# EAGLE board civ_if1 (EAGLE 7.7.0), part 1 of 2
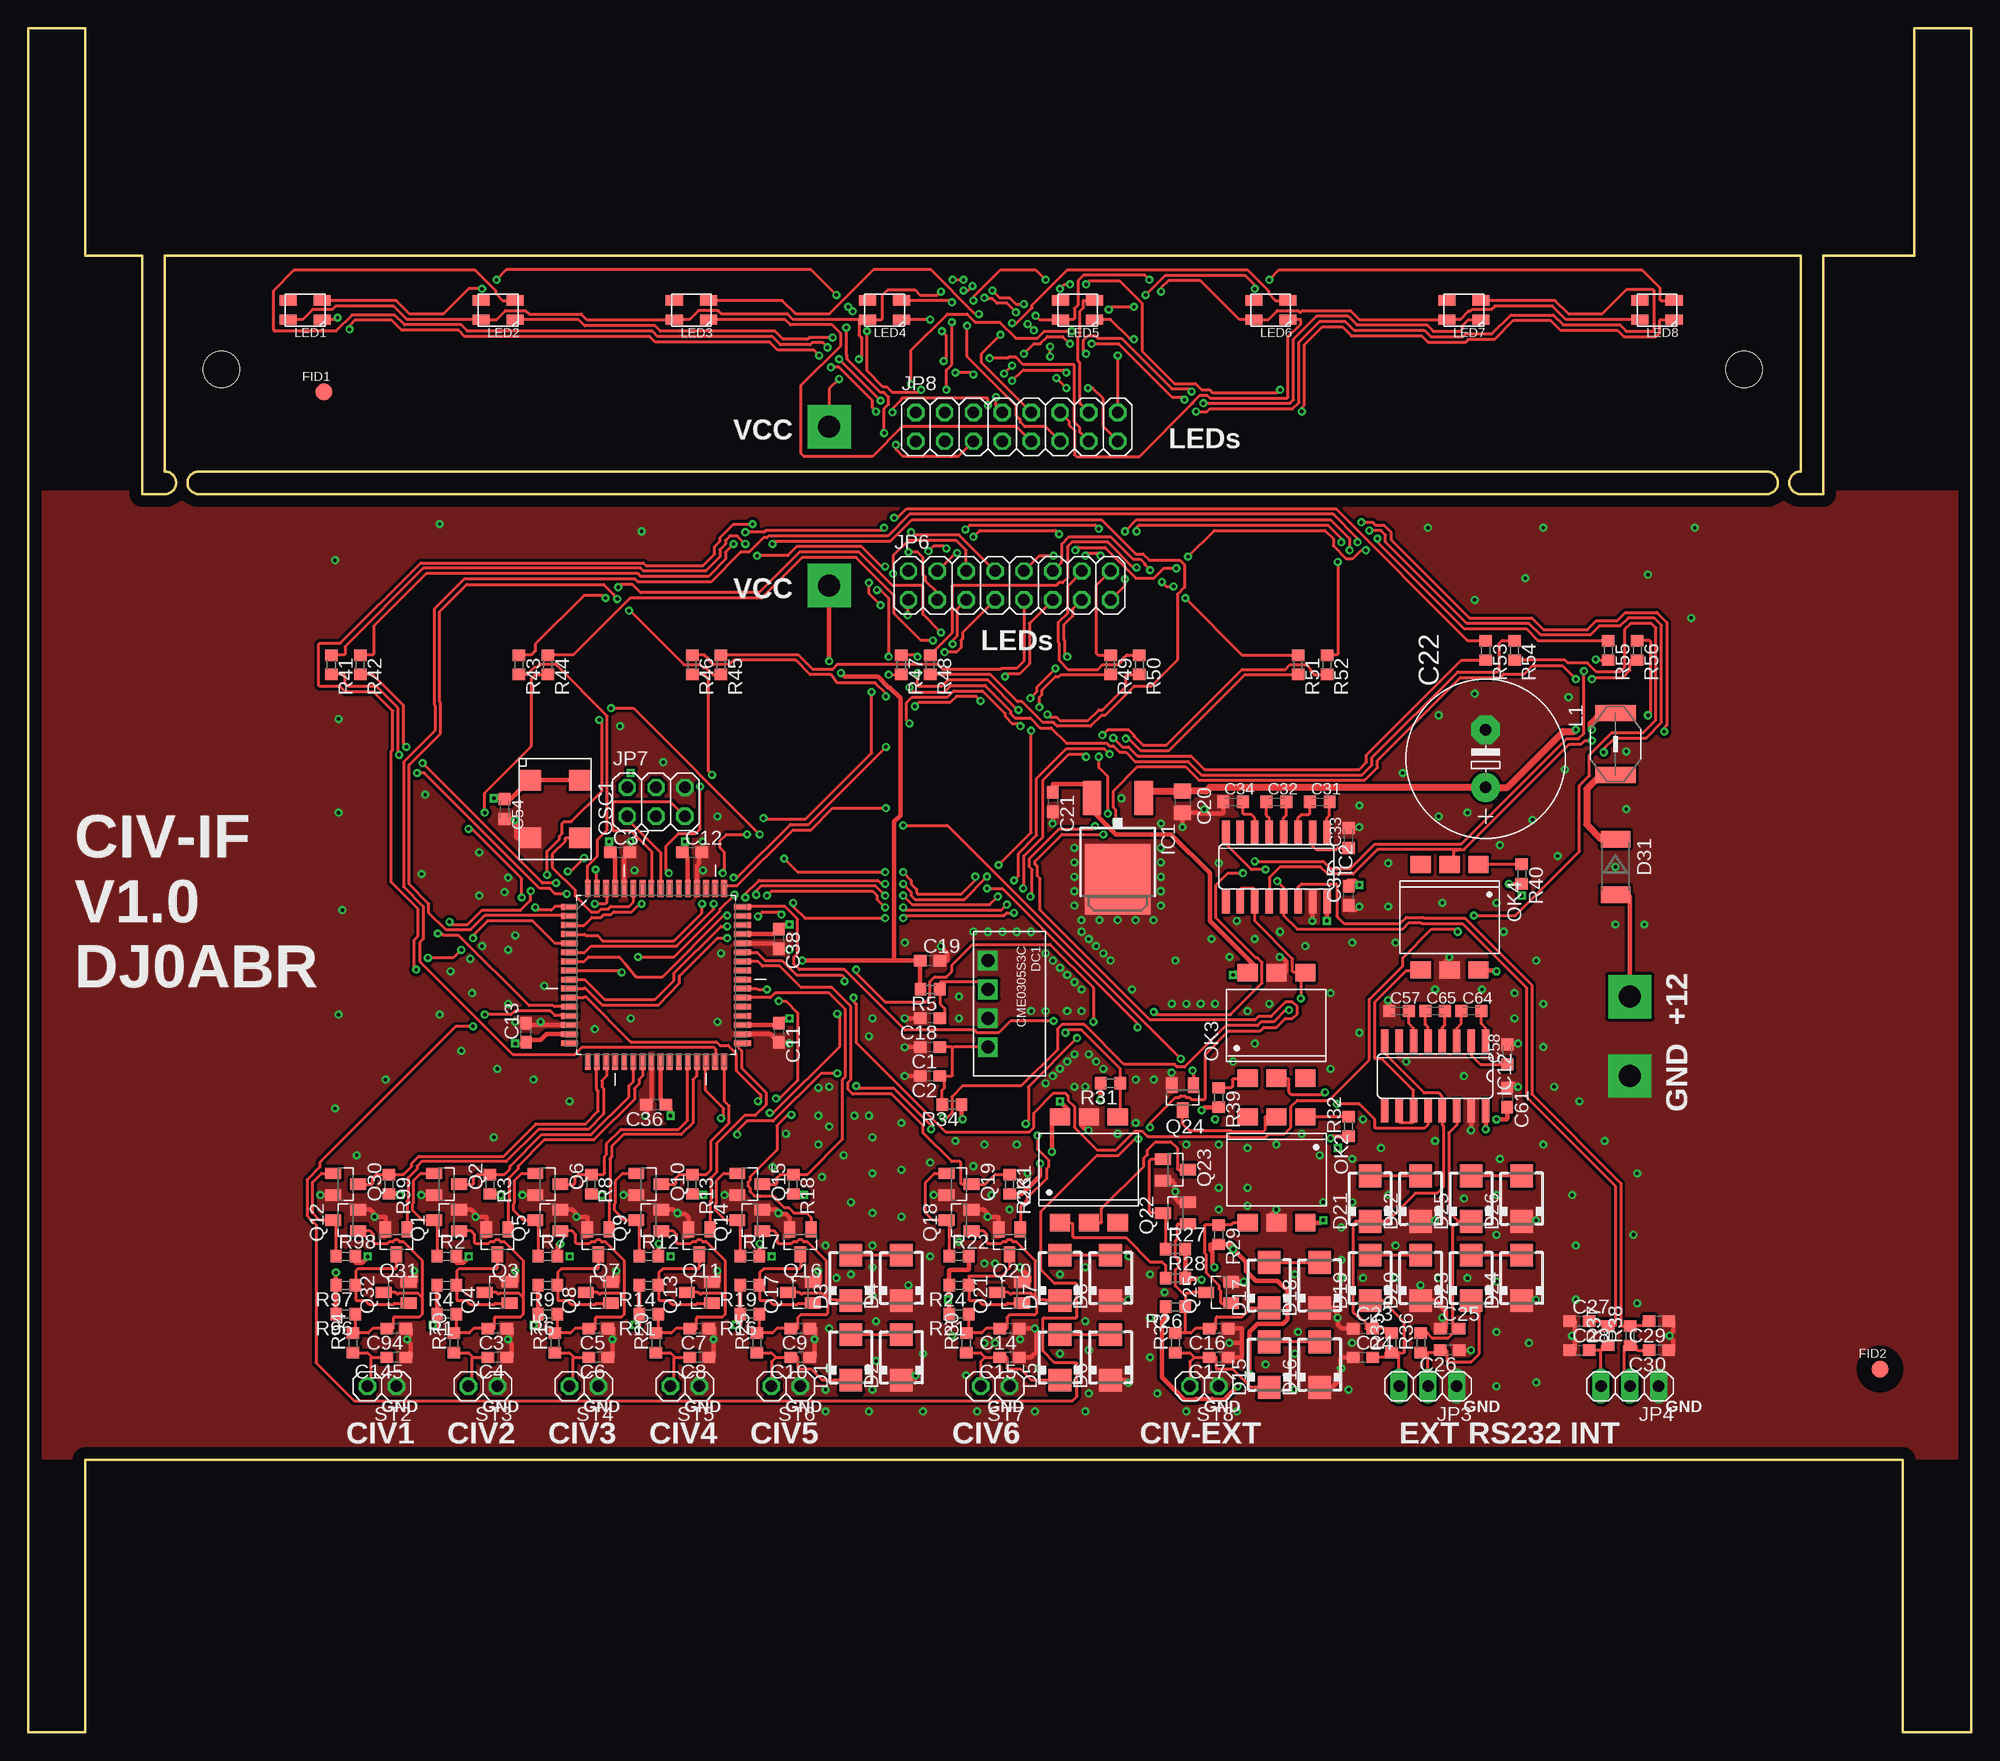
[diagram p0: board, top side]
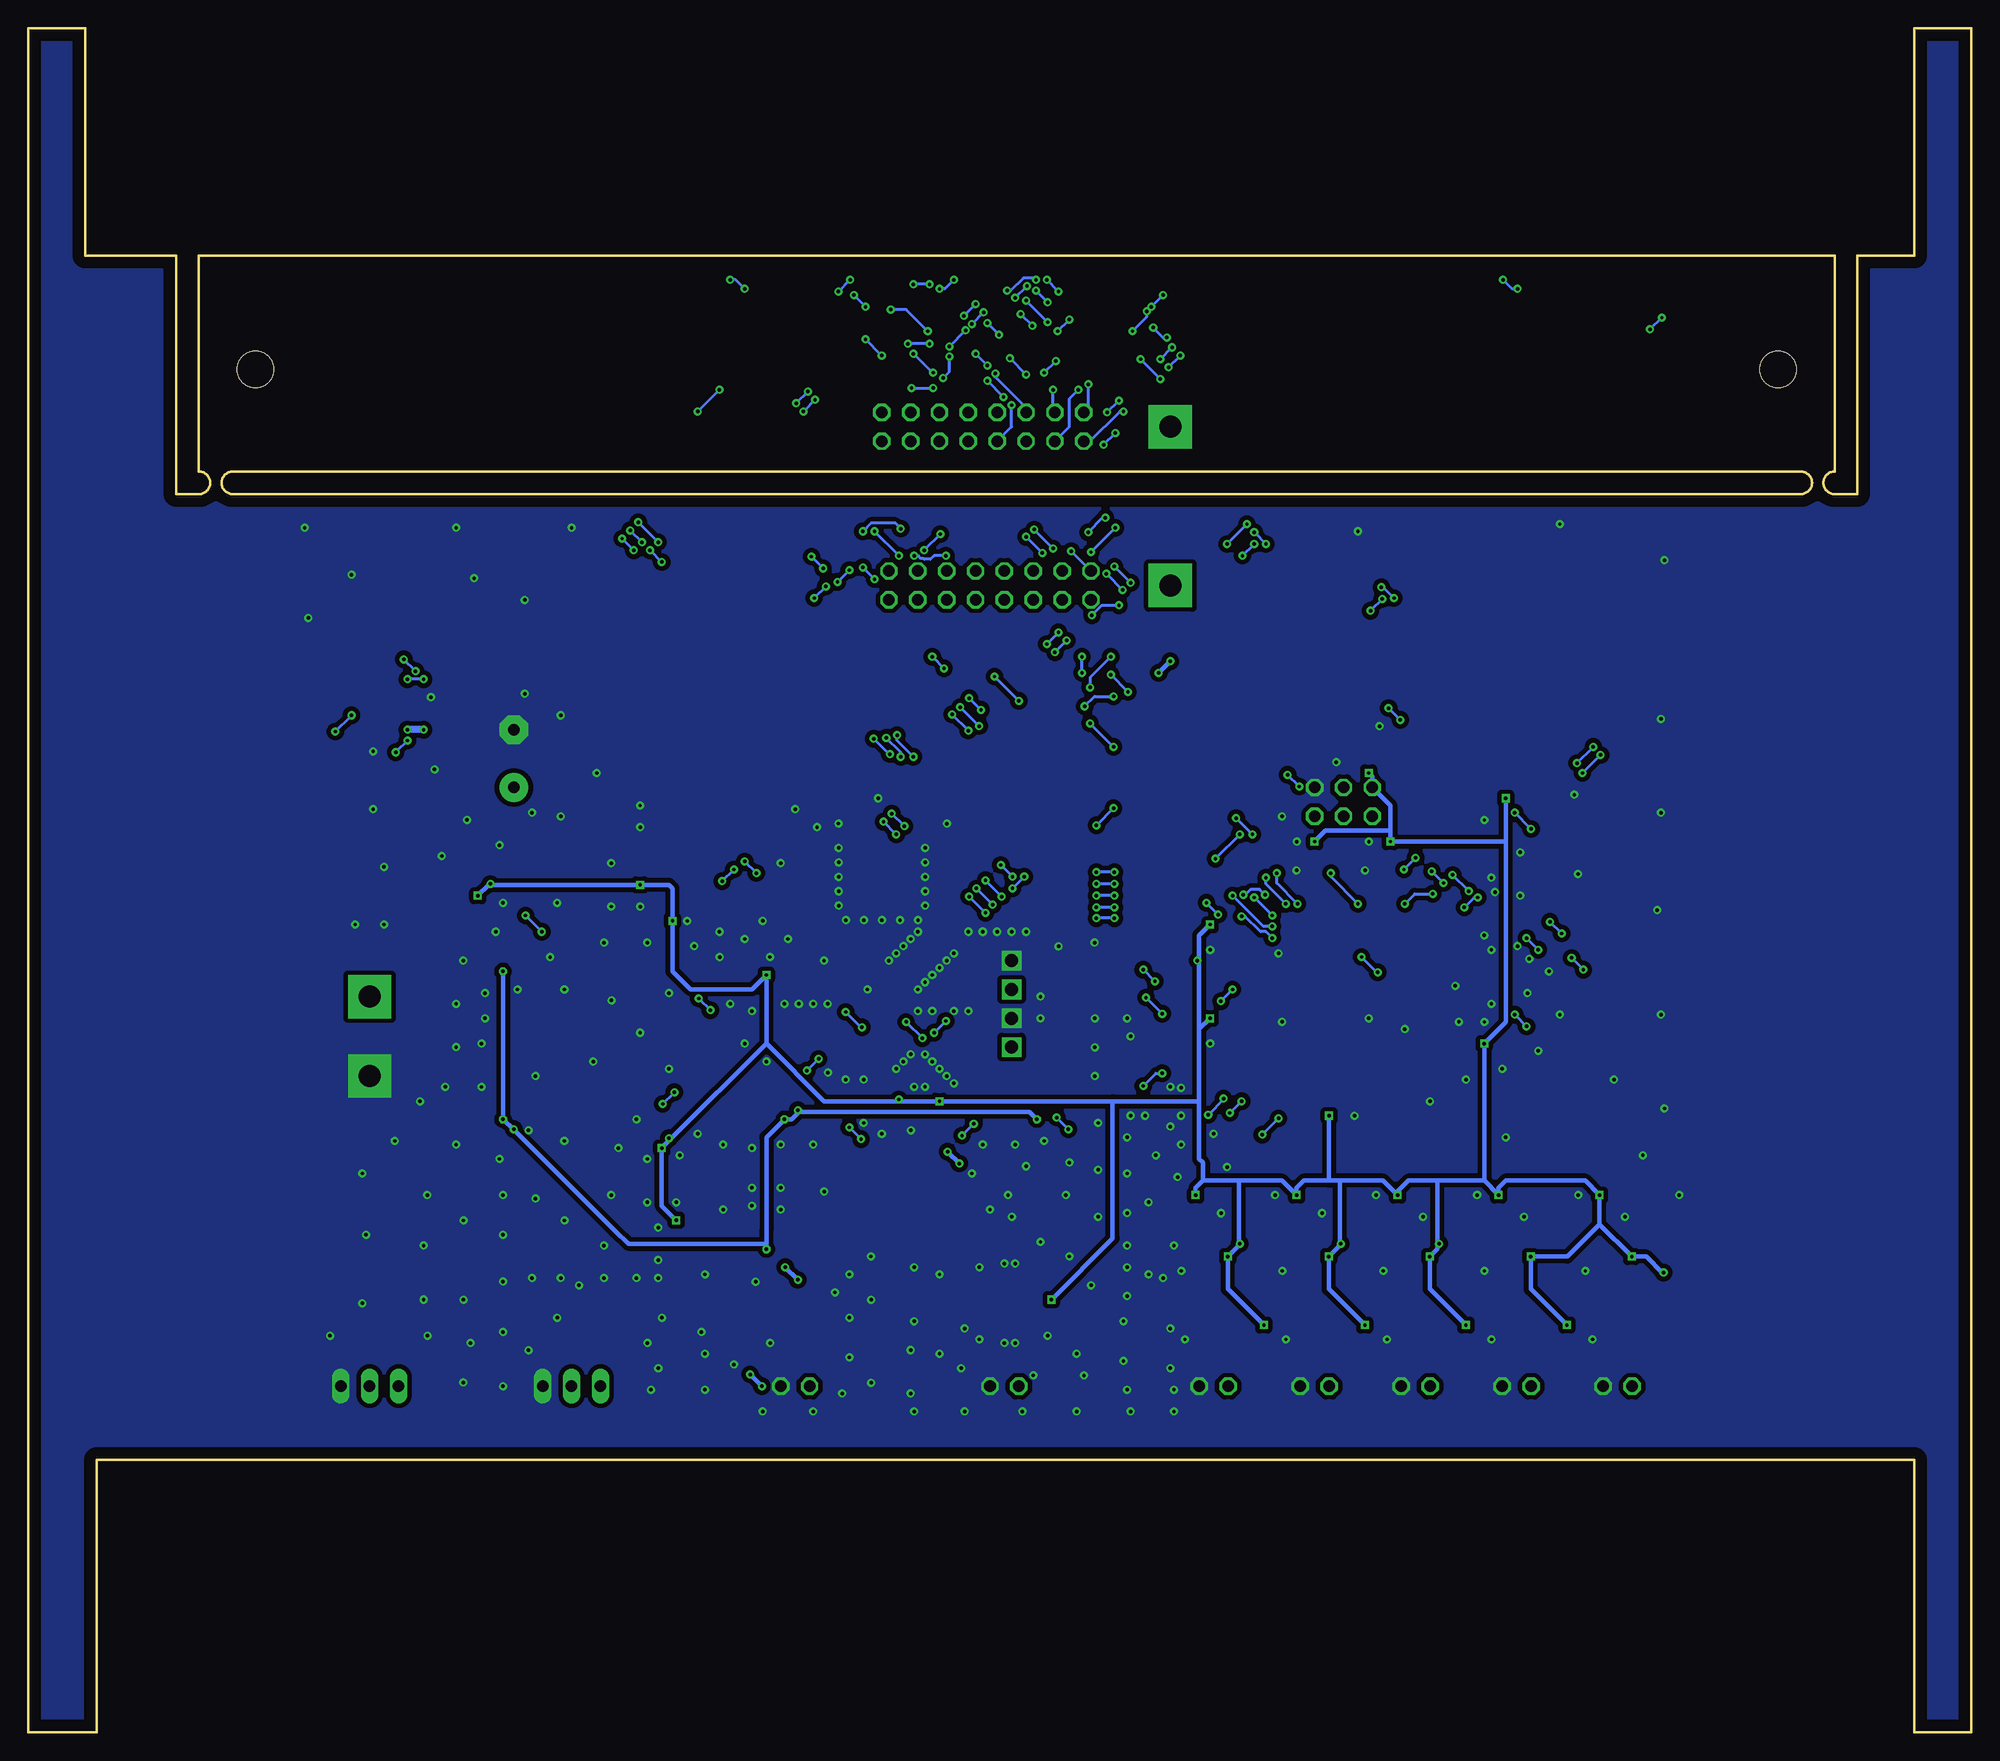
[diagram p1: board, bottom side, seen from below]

Size 171 x 150 mm. Coordinates in mm from the lower left corner, seen from the top.
Outline: 0,0 5,0 5,24 165,24 165,0 171,0 171,150 166,150 166,130 158,130 158,109 156,109 arc-180 156,111 156,130 12,130 12,111 arc-180 12,109 10,109 10,130 5,130 5,150 0,150 0,0
Outline: 153,111 15,111 arc180 15,109 153,109 arc180 153,111
Copper layers (1*16): Top 0.035mm / dielectric 1.5mm / Bottom 0.035mm
Design rules "default *": minimum track width 10mil, minimum drill 0.3mm, track to track 8mil, track to pad 8mil, pad to pad 8mil, via to via 8mil, smd to smd 0mil, copper to edge 40mil, drill to drill 8mil, minimum pad ring 10mil, minimum via ring 8mil, stop-mask expansion 4mil, vias tented up to drill 0.31mm, thermal gap 10mil
Net classes: 1 Supply: width 0.406 mm, drill 0.3 mm; 2 v12: width 0.61 mm, drill 0.3 mm
Holes 3.2 mm at 17,120 151,120

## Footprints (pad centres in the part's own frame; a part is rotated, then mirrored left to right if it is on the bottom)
C0603 = smd 1.1 x 1: 1 -0.85,0; 2 0.85,0
C0805 = smd 1.3 x 1.5: 1 -0.95,0; 2 0.95,0
E5-13 = drill 1.016 pad 2.54: + -2.54,0 | drill 1.016 pad 2.54 octagon: - 2.54,0
C0603K = smd 1.05 x 1.08: 1 -0.875,0; 2 0.875,0
SMA = smd 2 x 2: A 2,0; C -2,0
MELF = smd 1.45 x 2.6: 1 -2.445,0; 2 2.445,0
MURATA_DCDC = drill 1.15 square: 1 -3.81,0; 2 -1.27,0; 3 1.27,0; 4 3.81,0
FIDUCIAL = smd 1.5 x 1.5: P$1 0,0
DPACK = smd 1.6 x 3: 1 -2.28,-4.8; 3 2.28,-4.8 | smd 5.8 x 6.2: 4 0,2.38
SO16 = smd 0.66 x 2.032: 1 -4.445,-3.073; 2 -3.175,-3.073; 3 -1.905,-3.073; 4 -0.635,-3.073; 5 0.635,-3.073; 6 1.905,-3.073; 7 3.175,-3.073; 8 4.445,-3.073; 9 4.445,3.073; 10 3.175,3.073; 11 1.905,3.073; 12 0.635,3.073; 13 -0.635,3.073; 14 -1.905,3.073; 15 -3.175,3.073; 16 -4.445,3.073
THICKPIN = drill 1.93 pad 3.81 square: 1 0,0
1X03 = drill 1.016 long: 1 -2.54,0; 2 0,0; 3 2.54,0
2X08 = drill 1.016 octagon: 1 -8.89,-1.27; 2 -8.89,1.27; 3 -6.35,-1.27; 4 -6.35,1.27; 5 -3.81,-1.27; 6 -3.81,1.27; 7 -1.27,-1.27; 8 -1.27,1.27; 9 1.27,-1.27; 10 1.27,1.27; 11 3.81,-1.27; 12 3.81,1.27; 13 6.35,-1.27; 14 6.35,1.27; 15 8.89,-1.27; 16 8.89,1.27
2X03 = drill 1.016 octagon: 1 -2.54,-1.27; 2 -2.54,1.27; 3 0,-1.27; 4 0,1.27; 5 2.54,-1.27; 6 2.54,1.27
S = smd 1.4 x 3.56: 1 -2.73,0; 2 2.73,0
PLCC4_WE_LED = smd 1.5 x 0.9: 1 1.51,0.88; 2 1.51,-0.82; 3 -1.49,0.88; 4 -1.49,-0.82
DIL6-SMD = smd 1.78 x 1.52: 1 -2.54,-4.645; 2 0,-4.645; 3 2.54,-4.645; 4 2.54,4.645; 5 0,4.645; 6 -2.54,4.645
QOSC_AQO7015 = smd 1.8 x 2: 1 0,-0.318; 2 5.08,-0.318; 3 5.08,4.128; 4 0,4.128
SOT23 = smd 1 x 1.4: 1 -0.95,-1.1; 2 0.95,-1.1; 3 0,1.1
R0603 = smd 1 x 1.1: 1 -0.85,0; 2 0.85,0
PINHEAD1X2 = drill 1.016 octagon: 1 -1.27,0; 2 1.27,0
QFP80P1600X1600X120-64N = smd 1.473 x 0.508: 1 -7.62,5.994; 2 -7.62,5.207; 3 -7.62,4.394; 4 -7.62,3.607; 5 -7.62,2.794; 6 -7.62,2.007; 7 -7.62,1.194; 8 -7.62,0.406; 9 -7.62,-0.406; 10 -7.62,-1.194; 11 -7.62,-2.007; 12 -7.62,-2.794; 13 -7.62,-3.607; 14 -7.62,-4.394; 15 -7.62,-5.207; 16 -7.62,-5.994; 33 7.62,-5.994; 34 7.62,-5.207; 35 7.62,-4.394; 36 7.62,-3.607; 37 7.62,-2.794; 38 7.62,-2.007; 39 7.62,-1.194; 40 7.62,-0.406; 41 7.62,0.406; 42 7.62,1.194; 43 7.62,2.007; 44 7.62,2.794; 45 7.62,3.607; 46 7.62,4.394; 47 7.62,5.207; 48 7.62,5.994 | smd 0.508 x 1.473: 17 -5.994,-7.62; 18 -5.207,-7.62; 19 -4.394,-7.62; 20 -3.607,-7.62; 21 -2.794,-7.62; 22 -2.007,-7.62; 23 -1.194,-7.62; 24 -0.406,-7.62; 25 0.406,-7.62; 26 1.194,-7.62; 27 2.007,-7.62; 28 2.794,-7.62; 29 3.607,-7.62; 30 4.394,-7.62; 31 5.207,-7.62; 32 5.994,-7.62; 49 5.994,7.62; 50 5.207,7.62; 51 4.394,7.62; 52 3.607,7.62; 53 2.794,7.62; 54 2.007,7.62; 55 1.194,7.62; 56 0.406,7.62; 57 -0.406,7.62; 58 -1.194,7.62; 59 -2.007,7.62; 60 -2.794,7.62; 61 -3.607,7.62; 62 -4.394,7.62; 63 -5.207,7.62; 64 -5.994,7.62

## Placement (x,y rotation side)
C1  100n  [C0603]  79.38,60.33 180 top
C2  1u  [C0603]  79.38,57.78 180 top
C3  1n  [C0603]  41.27,35.56 180 top
C4  1n  [C0603]  41.27,33.02 180 top
C5  1n  [C0603]  50.16,35.56 180 top
C6  1n  [C0603]  50.16,33.02 180 top
C7  1n  [C0603]  59.05,35.56 180 top
C8  1n  [C0603]  59.05,33.02 180 top
C9  1n  [C0603]  67.94,35.56 180 top
C10  1n  [C0603]  67.94,33.02 180 top
C11  100n  [C0603]  66.04,61.59 270 top
C12  100n  [C0603]  58.42,77.47 0 top
C13  1u  [C0603]  43.81,61.59 90 top
C14  1n  [C0603]  86.36,35.56 180 top
C15  1n  [C0603]  86.36,33.02 180 top
C16  100p  [C0603]  104.78,35.56 180 top
C17  100p  [C0603]  104.78,33.02 180 top
C18  1u  [C0603]  79.38,62.87 180 top
C19  1u  [C0603]  79.38,67.94 0 top
C20  10u  [C0805]  101.6,81.92 270 top
C21  10u  [C0603]  90.17,81.92 270 top
C22  1000u/16  [E5-13]  128.27,85.72 90 top
C23  100p  [C0603]  117.47,35.56 0 top
C24  100p  [C0603]  117.47,33.02 0 top
C25  100p  [C0603]  125.09,35.56 0 top
C26  100p  [C0603]  125.09,33.66 180 top
C27  1n  [C0603]  136.53,36.2 0 top
C28  1n  [C0603]  136.53,33.66 0 top
C29  1n  [C0603]  143.51,36.2 180 top
C30  1n  [C0603]  143.51,33.66 180 top
C31  1u  [C0603K]  113.67,81.92 0 top
C32  1u  [C0603K]  109.86,81.92 0 top
C33  1u  [C0603K]  116.2,78.74 90 top
C34  1u  [C0603K]  106.05,81.92 0 top
C35  1u  [C0603]  116.2,73.66 90 top
C36  100n  [C0603]  55.24,55.24 180 top
C37  100n  [C0603]  52.07,77.47 0 top
C38  1u  [C0603]  66.04,69.85 270 top
C54  1u  [C0603K]  41.91,81.28 270 top
C57  1u  [C0603K]  120.65,63.5 0 top
C58  1u  [C0603K]  130.18,59.69 90 top
C61  1u  [C0603]  130.18,55.88 270 top
C64  1u  [C0603K]  127,63.5 0 top
C65  1u  [C0603K]  123.83,63.5 0 top
C94  1n  [C0603]  32.38,35.56 180 top
C145  1n  [C0603]  32.38,33.02 180 top
D1  SMBJ15A  [SMA]  72.39,33.02 90 top
D2  SMBJ15A  [SMA]  76.83,33.02 90 top
D3  SMBJ15A  [SMA]  72.39,40.01 90 top
D4  SMBJ15A  [SMA]  76.83,40.01 90 top
D5  SMBJ15A  [SMA]  90.81,33.02 90 top
D6  SMBJ15A  [SMA]  95.25,33.02 90 top
D7  SMBJ15A  [SMA]  90.81,40.01 90 top
D8  SMBJ15A  [SMA]  95.25,40.01 90 top
D15  SMBJ15A  [SMA]  109.22,32.38 90 top
D16  SMBJ15A  [SMA]  113.67,32.38 90 top
D17  SMBJ15A  [SMA]  109.22,39.37 90 top
D18  SMBJ15A  [SMA]  113.67,39.37 90 top
D19  SMBJ15A  [SMA]  118.11,40.01 90 top
D20  SMBJ15A  [SMA]  122.56,40.01 90 top
D21  SMBJ15A  [SMA]  118.11,46.99 90 top
D22  SMBJ15A  [SMA]  122.56,46.99 90 top
D23  SMBJ15A  [SMA]  127,40.01 90 top
D24  SMBJ15A  [SMA]  131.44,40.01 90 top
D25  SMBJ15A  [SMA]  127,46.99 90 top
D26  SMBJ15A  [SMA]  131.44,46.99 90 top
D31  1N4001  [MELF]  139.7,76.2 270 top
DC1  CME0305S3C  [MURATA_DCDC]  84.45,64.14 270 top
FID1  FIDUCIAL  [FIDUCIAL]  26,118 0 top
FID2  FIDUCIAL  [FIDUCIAL]  163,32 0 top
IC1  LF33CDT-DPAK  [DPACK]  95.89,77.47 180 top
IC2  MAX3232  [SO16]  109.86,76.2 180 top
IC12  MAX3232  [SO16]  123.83,57.78 180 top
JP1  [THICKPIN]  140.97,64.77 90 top
JP2  [THICKPIN]  140.97,57.78 90 top
JP3  [1X03]  123.19,30.48 180 top
JP4  [1X03]  140.97,30.48 180 top
JP5  [THICKPIN]  70.48,100.97 0 top
JP6  [2X08]  86.36,100.97 0 top
JP7  Program  [2X03]  55.24,81.92 0 top
JP8  [2X08]  87,114.94 0 top
JP9  [THICKPIN]  70.48,114.94 0 top
L1  WE74451147/47uH  [S]  139.7,87 270 top
LED1  RGBLED  [PLCC4_WE_LED]  24.36,125.24 180 top
LED2  RGBLED  [PLCC4_WE_LED]  41.37,125.24 180 top
LED3  RGBLED  [PLCC4_WE_LED]  58.37,125.24 180 top
LED4  RGBLED  [PLCC4_WE_LED]  75.36,125.24 180 top
LED5  RGBLED  [PLCC4_WE_LED]  92.36,125.24 180 top
LED6  RGBLED  [PLCC4_WE_LED]  109.36,125.24 180 top
LED7  RGBLED  [PLCC4_WE_LED]  126.36,125.24 180 top
LED8  RGBLED  [PLCC4_WE_LED]  143.37,125.24 180 top
OK1  H11L1SM  [DIL6-SMD]  93.34,49.53 0 top
OK2  H11L1SM  [DIL6-SMD]  109.86,49.53 180 top
OK3  H11L1SM  [DIL6-SMD]  109.86,62.23 0 top
OK4  H11L1SM  [DIL6-SMD]  125.09,71.75 180 top
OSC1  OSZ8MHz  [QOSC_AQO7015]  44.45,83.82 270 top
Q1  N-CH_MOSFET  [SOT23]  36.83,45.09 90 top
Q2  N-CH_MOSFET  [SOT23]  36.83,48.26 270 top
Q3  N-CH_MOSFET  [SOT23]  41.27,43.18 180 top
Q4  N-CH_MOSFET  [SOT23]  41.27,38.73 90 top
Q5  N-CH_MOSFET  [SOT23]  45.72,45.09 90 top
Q6  N-CH_MOSFET  [SOT23]  45.72,48.26 270 top
Q7  N-CH_MOSFET  [SOT23]  50.16,43.18 180 top
Q8  N-CH_MOSFET  [SOT23]  50.16,38.73 90 top
Q9  N-CH_MOSFET  [SOT23]  54.61,45.09 90 top
Q10  N-CH_MOSFET  [SOT23]  54.61,48.26 270 top
Q11  N-CH_MOSFET  [SOT23]  59.05,43.18 180 top
Q12  N-CH_MOSFET  [SOT23]  27.94,45.09 90 top
Q13  N-CH_MOSFET  [SOT23]  59.05,38.73 90 top
Q14  N-CH_MOSFET  [SOT23]  63.5,45.09 90 top
Q15  N-CH_MOSFET  [SOT23]  63.5,48.26 270 top
Q16  N-CH_MOSFET  [SOT23]  67.94,43.18 180 top
Q17  N-CH_MOSFET  [SOT23]  67.94,38.73 90 top
Q18  N-CH_MOSFET  [SOT23]  81.92,45.09 90 top
Q19  N-CH_MOSFET  [SOT23]  81.92,48.26 270 top
Q20  N-CH_MOSFET  [SOT23]  86.36,43.18 180 top
Q21  N-CH_MOSFET  [SOT23]  86.36,38.73 90 top
Q22  N-CH_MOSFET  [SOT23]  100.97,45.72 90 top
Q23  N-CH_MOSFET  [SOT23]  100.97,49.53 270 top
Q24  N-CH_MOSFET  [SOT23]  101.6,55.88 180 top
Q25  N-CH_MOSFET  [SOT23]  104.78,38.73 90 top
Q30  N-CH_MOSFET  [SOT23]  27.94,48.26 270 top
Q31  N-CH_MOSFET  [SOT23]  32.38,43.18 180 top
Q32  N-CH_MOSFET  [SOT23]  32.38,38.73 90 top
R1  10k  [R0603]  36.83,36.83 180 top
R2  10k  [R0603]  36.83,41.91 0 top
R3  10k  [R0603]  40.64,48.26 270 top
R4  10k  [R0603]  36.83,39.37 180 top
R5  1kOhm-Ferr  [R0603]  79.38,65.41 180 top
R6  10k  [R0603]  45.72,36.83 180 top
R7  10k  [R0603]  45.72,41.91 0 top
R8  10k  [R0603]  49.53,48.26 270 top
R9  10k  [R0603]  45.72,39.37 180 top
R10  1kOhm-Ferr  [R0603]  37.47,34.29 90 top
R11  10k  [R0603]  54.61,36.83 180 top
R12  10k  [R0603]  54.61,41.91 0 top
R13  10k  [R0603]  58.42,48.26 270 top
R14  10k  [R0603]  54.61,39.37 180 top
R15  1kOhm-Ferr  [R0603]  46.35,34.29 90 top
R16  10k  [R0603]  63.5,36.83 180 top
R17  10k  [R0603]  63.5,41.91 0 top
R18  10k  [R0603]  67.31,48.26 270 top
R19  10k  [R0603]  63.5,39.37 180 top
R20  1kOhm-Ferr  [R0603]  55.24,34.29 90 top
R21  10k  [R0603]  81.92,36.83 180 top
R22  10k  [R0603]  81.92,41.91 0 top
R23  10k  [R0603]  86.36,48.26 270 top
R24  10k  [R0603]  81.92,39.37 180 top
R25  1kOhm-Ferr  [R0603]  64.14,34.29 90 top
R26  10k  [R0603]  100.97,37.47 180 top
R27  10k  [R0603]  100.97,42.55 0 top
R28  680  [R0603]  100.97,40.01 0 top
R29  1k  [R0603]  104.78,43.81 270 top
R30  1kOhm-Ferr  [R0603]  82.55,34.29 90 top
R31  1k  [R0603]  95.25,57.15 180 top
R32  330  [R0603]  116.2,53.34 90 top
R33  1kOhm-Ferr  [R0603]  100.97,34.29 90 top
R34  1kOhm-Ferr  [R0603]  81.28,55.24 180 top
R35  1kOhm-Ferr  [R0603]  120.02,34.29 90 top
R36  1kOhm-Ferr  [R0603]  122.56,34.29 90 top
R37  1kOhm-Ferr  [R0603]  139.06,34.92 90 top
R38  1kOhm-Ferr  [R0603]  140.97,34.92 90 top
R39  680  [R0603]  104.78,55.88 270 top
R40  330  [R0603]  131.44,75.56 270 top
R41  2k2  [R0603]  26.67,93.98 270 top
R42  680  [R0603]  29.21,93.98 270 top
R43  2k2  [R0603]  43.18,93.98 270 top
R44  680  [R0603]  45.72,93.98 270 top
R45  2k2  [R0603]  60.96,93.98 270 top
R46  680  [R0603]  58.42,93.98 270 top
R47  2k2  [R0603]  76.83,93.98 270 top
R48  680  [R0603]  79.38,93.98 270 top
R49  2k2  [R0603]  95.25,93.98 270 top
R50  680  [R0603]  97.79,93.98 270 top
R51  2k2  [R0603]  111.76,93.98 270 top
R52  680  [R0603]  114.3,93.98 270 top
R53  2k2  [R0603]  128.27,95.25 270 top
R54  680  [R0603]  130.81,95.25 270 top
R55  2k2  [R0603]  139.06,95.25 270 top
R56  680  [R0603]  141.6,95.25 270 top
R94  1kOhm-Ferr  [R0603]  28.57,34.29 90 top
R96  10k  [R0603]  27.94,36.83 180 top
R97  10k  [R0603]  27.94,39.37 180 top
R98  10k  [R0603]  27.94,41.91 0 top
R99  10k  [R0603]  31.75,48.26 270 top
ST2  [PINHEAD1X2]  31.11,30.48 180 top
ST3  [PINHEAD1X2]  40.01,30.48 180 top
ST4  [PINHEAD1X2]  48.9,30.48 180 top
ST5  [PINHEAD1X2]  57.78,30.48 180 top
ST6  [PINHEAD1X2]  66.67,30.48 180 top
ST7  [PINHEAD1X2]  85.09,30.48 180 top
ST8  [PINHEAD1X2]  103.5,30.48 180 top
U1  ATXMEGA256A3-AU  [QFP80P1600X1600X120-64N]  55.24,66.67 0 top

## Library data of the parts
C1-C38 C54 C57 C58 C61 C64 C65 C94 C145 R1-R56 R94 R96-R99 = rcl
D1-D8 D15-D26 D31 DC1 FID1 FID2 JP1 JP2 JP5 JP9 LED1-LED8 OSC1 Q1-Q25 Q30-Q32 ST2-ST8 = km
IC1 = v-reg
IC2 IC12 = maxim; MPN: MAX3232CSE; OC_FARNELL: 9725490; OC_NEWARK: 90C2890
JP3 JP4 JP6-JP8 = pinhead
L1 = WE-PD3; MPN: 74451147; OC_FARNELL: 1636065; OC_NEWARK: 08P2637; PACKAGE: Type S; SUPPLIER: Würth Elektronik eiSos GmbH
OK1-OK4 = optocoupler; OC_FARNELL: unknown; OC_NEWARK: unknown
U1 = ATXMEGA256A3-AU; DESCRIPTION: MCU; MPN: ATXMEGA256A3-AU; OC_FARNELL: 1748554; OC_NEWARK: -; PACKAGE: QFP-64; SUPPLIER: Atmel

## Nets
GND [Supply]: C1.2 C2.2 C3.1 C4.1 C5.1 C6.1 C7.1 C8.1 C9.1 C10.1 C11.2 C12.2 C13.2 C14.1 C15.1 C16.1 C17.1 C18.2 C19.2 C20.2 C21.2 C22.- C23.1 C24.1 C25.1 C26.1 C27.1 C28.1 C29.1 C30.1 C33.2 C34.1 C35.1 C36.2 C37.2 C38.2 C54.2 C57.1 C58.2 C61.1 C94.1 C145.1 D2.C D4.C D6.C D8.C D16.C D18.C D20.C D22.C D24.C D26.C DC1.1 DC1.3 IC1.4 IC2.15 IC12.15 JP2.1 JP3.1 JP4.1 JP7.6 OK1.5 OK2.5 OK3.5 OK4.5 OSC1.2 Q1.2 Q2.2 Q3.2 Q4.2 Q5.2 Q6.2 Q7.2 Q8.2 Q9.2 Q10.2 Q11.2 Q12.2 Q13.2 Q14.2 Q15.2 Q16.2 Q17.2 Q18.2 Q19.2 Q20.2 Q21.2 Q22.2 Q23.2 Q24.2 Q25.2 Q30.2 Q31.2 Q32.2 ST2.1 ST3.1 ST4.1 ST5.1 ST6.1 ST7.1 ST8.1 U1.14 U1.24 U1.34 U1.44 U1.52 U1.60
N$1: OK1.2 Q23.3
N$2: Q1.3 Q2.1 R2.1
N$3: OSC1.3 U1.59
N$4: C1.1 C2.1 DC1.4 R34.2
N$5: Q3.3 Q4.1 R4.1
N$6: C18.1 DC1.2 R5.1
N$7: C4.2 R10.1 ST3.2
N$8: OK2.1 R32.2
N$9: Q5.3 Q6.1 R7.1
N$10: C94.2 Q12.1 Q32.3 R94.2 R96.1
N$11: C3.2 Q1.1 Q4.3 R1.1 R10.2
N$12: Q7.3 Q8.1 R9.1
N$13: C6.2 R15.1 ST4.2
N$14: C5.2 Q5.1 Q8.3 R6.1 R15.2
N$15: C8.2 R20.1 ST5.2
N$16: Q9.3 Q10.1 R12.1
N$17: Q22.3 Q23.1 R27.1
N$18: OK2.4 Q25.1 R29.1
N$19: Q11.3 Q13.1 R14.1
N$20 [v12]: C20.1 C22.+ IC1.1 L1.1
N$21: C7.2 Q9.1 Q13.3 R11.1 R20.2
N$22: C10.2 D1.C R25.1 ST6.2
N$23: Q14.3 Q15.1 R17.1
N$24: C9.2 D3.C Q14.1 Q17.3 R16.1 R25.2
N$25: C15.2 D5.C R30.1 ST7.2
N$26: Q16.3 Q17.1 R19.1
N$27: JP6.1 R41.1
N$28: C14.2 D7.C Q18.1 Q21.3 R21.1 R30.2
N$29: C17.2 D15.C R33.1 ST8.2
N$30: Q18.3 Q19.1 R22.1
N$31: C16.2 D17.C Q22.1 Q25.3 R26.1 R33.2
N$32: JP6.3 R42.1
N$33: Q20.3 Q21.1 R24.1
N$34 [Supply]: D31.2 JP1.1
N$35: D15.A D16.A
N$36: D17.A D18.A
N$37: C24.2 D19.C JP3.3 R35.1
N$38: C23.2 D21.C IC12.8 IC12.13 R35.2
N$39: D19.A D20.A
N$40: D21.A D22.A
N$41: C26.2 D23.C JP3.2 R36.1
N$42: C28.2 JP4.3 R37.1
N$43: D23.A D24.A
N$44: D25.A D26.A
N$45: C64.1 IC12.3
N$46: C64.2 IC12.1
N$47: C65.2 IC12.4
N$48: C65.1 IC12.5
N$49: C58.1 IC12.2
N$50: C57.2 IC12.6
N$51: IC12.10 IC12.11 OK4.4
N$52: IC12.12 OK3.2
N$53: C27.2 IC2.8 IC2.13 R37.2
N$54: C25.2 D25.C IC12.14 R36.2
N$55: JP6.5 R43.1
N$56: JP6.7 R44.1
N$57: C30.2 JP4.2 R38.1
N$58: JP6.9 R45.1
N$59: JP6.11 R46.1
N$60: C31.1 IC2.3
N$61: C31.2 IC2.1
N$62: C32.2 IC2.4
N$63: C32.1 IC2.5
N$64: C33.1 IC2.2
N$65: C34.2 IC2.6
N$66: IC2.10 IC2.11 OK3.4 U1.30
N$67: IC2.12 OK4.2 U1.31
N$68: C29.2 IC2.14 R38.2
N$69: JP6.13 R47.1
N$70: OK3.1 R39.1
N$71: OK4.1 R40.1
N$72: JP6.15 R48.1
N$73: JP6.16 R49.1
N$74: JP6.14 R50.1
N$75: JP6.12 R51.1
N$76: JP6.10 R52.1
N$77: JP6.8 R53.1
N$78: JP6.6 R54.1
N$79: JP6.4 R55.1
N$80: JP6.2 R56.1
N$81: R41.2 U1.62
N$82: R42.2 U1.63
N$83: R43.2 U1.64
N$84: R44.2 U1.1
N$85: R45.2 U1.2
N$86: R46.2 U1.3
N$87: R47.2 U1.4
N$88: R48.2 U1.5
N$89: R49.2 U1.6
N$90: R50.2 U1.7
N$91: R51.2 U1.8
N$92: R52.2 U1.9
N$93: R53.2 U1.10
N$94: R54.2 U1.11
N$95 [v12]: D31.1 L1.2
N$96: R55.2 U1.12
N$97: R56.2 U1.13
N$98: D1.A D2.A
N$99: Q12.3 Q30.1 R98.1
N$100: JP7.5 U1.57
N$101: JP7.1 U1.56
N$102: D3.A D4.A
N$103: D5.A D6.A
N$104: D7.A D8.A
N$105: Q31.3 Q32.1 R97.1
N$106: C145.2 R94.1 ST2.2
N$107: OK2.2 Q24.3
N$108: JP9.1 LED1.1 LED2.1 LED3.1 LED4.1 LED5.1 LED6.1 LED7.1 LED8.1
N$109: JP8.1 LED1.3
N$110: JP8.3 LED1.4
N$111: JP8.5 LED2.3
N$112: JP8.7 LED2.4
N$113: JP8.9 LED3.3
N$114: JP8.11 LED3.4
N$115: JP8.13 LED4.3
N$116: JP8.15 LED4.4
N$117: JP8.16 LED5.3
N$118: JP8.14 LED5.4
N$119: JP8.12 LED6.3
N$120: JP8.10 LED6.4
N$121: JP8.8 LED7.3
N$122: JP8.6 LED7.4
N$123: JP8.4 LED8.3
N$124: JP8.2 LED8.4
PLUS-CIV [Supply]: C61.2 IC12.16 OK4.6 R26.2 R27.2 R28.2 R29.2 R34.1 R39.2
UART1: Q30.3 R99.1 U1.18
UART2: Q31.1 U1.19
UART3: Q2.3 R3.1 U1.22
UART4: Q3.1 U1.23
UART5: Q6.3 R8.1 U1.28
UART6: Q7.1 U1.29
UART7: Q10.3 R13.1 U1.32
UART8: Q11.1 U1.33
UART9: Q15.3 R18.1 U1.38
UART10: Q16.1 U1.39
UART11: Q19.3 R23.1 U1.42
UART12: Q20.1 U1.43
UART13: OK1.4 R31.1 U1.48
UART14: Q24.1 U1.49
UART15: OK1.1 R28.1
VCC [Supply]: C11.1 C12.1 C13.1 C19.1 C21.1 C35.2 C36.1 C37.1 C38.1 C54.1 IC1.3 IC2.16 JP5.1 JP7.2 OK1.6 OK2.6 OK3.6 OSC1.1 OSC1.4 R1.2 R2.2 R3.2 R4.2 R5.2 R6.2 R7.2 R8.2 R9.2 R11.2 R12.2 R13.2 R14.2 R16.2 R17.2 R18.2 R19.2 R21.2 R22.2 R23.2 R24.2 R31.2 R32.1 R40.2 R96.2 R97.2 R98.2 R99.2 U1.15 U1.25 U1.35 U1.45 U1.53 U1.61

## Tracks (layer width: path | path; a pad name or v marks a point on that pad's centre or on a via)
GND  (via drill 0.3)
  Top 0.406: U1.60 52.45,77 C37.2 53.01,77.56 v53.01,78.41 | U1.52 58.85,76.31 59.05,76.52 59.05,77.25 C12.2 59.35,77.56 v59.35,78.41 | U1.44 65.57,69.47 C38.2 66.15,68.89 v66.97,68.89 | U1.34 65.32,61.47 C11.2 66.89,60.74 66.99,60.64 66.98,60.64 v66.97,60.63 | U1.24 54.84,55.69 C36.2 54.4,54.4 v54.27,54.28 | U1.14 43.98,62.28 C13.2 43.72,62.54 v42.84,62.54 | C34.1 105.17,80.96 105.09,80.88 102.95,80.88 102.87,80.96 C20.2 101.6,79.69 v101.58,79.68 | C15.1 88.27,33.02 88.74,33.5 88.74,35.24 88.42,35.56 C14.1 87.31,35.4 87.31,34.61 v87.3,34.6 | C17.1 106.76,33.02 106.84,33.1 106.84,34.29 | 106.84,34.29 106.84,35.48 106.76,35.56 C16.1 | OK2.5 109.86,44.85 109.38,44.85 109.38,45.56 109.78,45.96 v109.84,46.03 | C54.2 42.7,80.41 42.78,80.33 v42.84,80.32 42.94,80.17 42.94,78.82 43.02,78.74 OSC1.2 | C57.1 119.78,64.29 119.7,64.37 v119.68,64.44 | C58.2 131.05,60.56 v131.11,60.63 | C33.2 117.08,79.61 v117.14,79.68 | C145.1 33.66,33.02 33.66,34.21 33.34,34.53 v33.32,34.6 33.42,34.77 33.66,35 33.66,35.56 C94.1 | C4.1 42.55,33.02 42.55,34.21 42.23,34.53 v42.21,34.6 42.31,34.77 42.55,35 42.55,35.56 C3.1 | C6.1 51.44,33.02 51.44,34.53 v51.42,34.6 51.51,34.77 51.51,35.56 C5.1 | C8.1 60.33,33.02 60.33,34.53 v60.31,34.6 60.4,34.77 60.4,35.56 C7.1 | C10.1 69.22,33.02 69.22,34.53 v69.2,34.6 69.29,34.77 69.29,35.56 C9.1 | C2.2 77.15,57.78 v77.14,57.78 | C1.2 77.15,60.33 v77.14,60.32 | C18.2 77.15,62.87 v77.14,62.86 | C19.2 80.88,67.94 80.88,68.58 80.33,69.14 v80.31,69.21 | C24.1 115.57,33.02 115.49,32.94 115.49,32.07 v115.55,32.06 115.41,31.91 115.41,31.04 114.78,30.4 113.67,30.4 D16.C
  Top 0.406: C23.1 115.57,35.56 115.25,35.88 115.25,36.43 v115.23,36.5 115.17,36.67 115.17,36.99 114.78,37.39 113.67,37.39 D18.C | C26.1 126.92,33.66 v126.98,33.65 | C25.1 124.78,35.56 124.78,36.12 124.46,36.43 v124.44,36.5 124.78,36.35 124.78,37.07 123.83,38.02 122.56,38.02 D20.C | C28.1 136.13,33.66 136.13,34.61 135.89,34.85 v135.87,34.92 135.97,35.08 136.13,35.24 136.13,36.2 C27.1 | C21.2 90.17,80.01 v90.15,80 | C30.1 144.78,33.66 144.78,34.53 144.46,34.85 v144.44,34.92 144.54,35.08 144.78,35.32 144.78,36.2 C29.1 | C35.1 116.2,72.39 116.84,72.39 117.08,72.63 v117.14,72.7 | C61.1 130.18,57.15 130.73,57.15 131.05,56.83 v131.11,56.82 | Q30.2 25.72,47.31 v25.7,47.3 | Q32.2 33.5,39.69 34.13,39.69 34.13,40.4 33.97,40.56 v33.95,40.63 | Q12.2 30.08,46.04 30.4,45.72 30.4,45.4 v30.46,45.39 30.64,45.4 31.35,45.4 31.43,45.32 Q31.2 | Q4.2 43.02,39.69 43.02,40.4 42.86,40.56 v42.84,40.63 | Q1.2 37.94,46.04 38.97,46.04 39.29,45.72 39.29,45.4 v39.35,45.39 39.53,45.4 40.24,45.4 40.32,45.32 Q3.2 | Q2.2 34.61,47.31 v34.59,47.3 | Q6.2 43.5,47.31 v43.48,47.3 | Q8.2 51.91,39.69 51.91,40.4 51.75,40.56 v51.73,40.63 | Q5.2 46.83,46.04 47.86,46.04 48.18,45.72 48.18,45.4 v48.24,45.39 48.42,45.4 49.13,45.4 49.21,45.32 Q7.2 | Q13.2 60.8,39.69 60.8,40.4 60.64,40.56 v60.62,40.63 | Q9.2 56.75,46.04 57.07,45.72 v57.13,45.71 57.31,45.64 57.78,45.64 58.1,45.32 Q11.2 | Q10.2 52.39,47.31 v52.37,47.3 | Q15.2 61.28,47.31 v61.26,47.3 | Q17.2 69.06,39.69 69.69,39.69 69.69,40.4 69.53,40.56 v69.52,40.63 | Q14.2 64.61,46.04 65.88,46.04 66.12,45.8 66.04,45.72 v66.02,45.71 66.2,45.64 66.67,45.64 66.99,45.32 Q16.2
  Top 0.406: Q19.2 80.8,47.31 79.69,47.31 v79.67,47.3 | Q21.2 87.47,39.69 88.11,39.69 88.11,40.08 87.31,40.88 v87.3,40.95 | Q18.2 84.06,46.04 84.38,45.72 84.38,45.4 v84.44,45.39 84.61,45.4 85.33,45.4 85.41,45.32 Q20.2 | Q25.2 106.92,39.69 v106.98,39.68 | Q22.2 102,46.67 101.28,46.67 100.97,46.99 100.97,47.55 v100.95,47.62 100.89,47.78 100.89,48.34 100.65,48.58 99.93,48.58 Q23.2 | Q24.2 100.65,58.02 v100.63,58.09 | OK1.5 93.34,54.21 92.63,54.21 92.63,53.5 93.19,52.94 93.27,52.94 v93.33,53.01 | OK3.5 109.86,66.91 110.65,66.91 110.73,66.99 110.73,67.87 110.25,68.34 110.17,68.26 v110.16,68.25 | OK4.5 125.09,67.07 124.62,67.07 124.62,67.79 125.02,68.18 v125.08,68.25 | D2.C 76.83,31.04 77.95,31.04 78.03,31.11 78.03,31.35 v78.09,31.42 | D4.C 76.83,38.02 77.47,38.02 77.47,39.29 v77.45,39.36 | D6.C 95.25,31.04 96.52,31.04 96.76,30.8 v96.82,30.79 | D8.C 95.25,38.02 96.76,38.02 v96.82,38.09 | D24.C 131.44,38.02 132.64,38.02 v132.7,38.09 | D22.C 122.56,45.01 123.75,45.01 v123.81,45.08 | D26.C 131.44,45.01 132.64,45.01 v132.7,45.08 | IC12.15 127,53.02 v126.98,53.01 | IC2.15 113.03,71.44 v113.01,71.43 | 106.84,34.29 105.73,34.29 v105.71,34.28
  Bottom 0.406: 109.86,46.04 v109.84,46.03
  other vias: 92.69,71.51 94.28,71.51 95.87,71.51 97.45,71.51 99.04,71.51 99.68,72.78 99.68,74.05 99.68,75.32 99.68,76.59 99.68,77.86 92.06,72.78 92.06,74.05 92.06,75.32 92.06,76.59 92.06,77.86 116.5,34.28 122.54,39.36 92.71,70.48 93.34,69.85 93.98,69.22 94.61,68.58 95.25,67.94 89.53,68.58 90.17,67.94 90.81,67.31 91.44,66.67 92.08,66.04 92.71,65.41 88.27,70.48 87,70.48 85.72,70.48 84.45,70.48 83.19,70.48 81.92,64.77 81.92,62.87 92.71,63.5 91.44,63.5 89.53,63.5 88.27,63.5 89.53,57.15 90.17,57.78 90.81,58.42 91.44,59.05 92.08,59.69 93.34,59.69 93.98,59.05 94.61,58.42 93.03,56.83 92.08,56.83 95.89,52.7 97.47,53.66 100.65,64.14 101.92,64.14 103.19,64.14 104.46,64.14 105.73,68.26 104.14,69.85 97.16,65.41 100.97,67.94 107.31,63.5 109.22,64.14 106.36,71.44 107.95,69.85 97.47,57.47 99.06,57.47 101.92,51.75 104.78,51.75 107.31,51.44 109.86,51.75 112.08,52.7 113.67,50.8 107.31,47.94 104.78,47.94 104.78,46.04 107.31,46.35 113.98,46.67 116.52,46.67 116.52,50.48 115.57,44.45 115.57,41.59 115.57,40.01 117.47,40.01 111.44,40.32 111.76,35.24 111.44,33.34 108.9,32.38 111.44,30.16 116.2,30.16 96.84,41.91 98.74,40.32 100.01,38.73 98.74,36.51 98.74,33.02 99.38,29.84 93.34,29.84 93.34,33.66 93.03,36.2 93.03,40.96 90.81,40.32 90.81,33.34 88.9,32.07 88.58,35.56 84.14,34.29 85.09,34.29 81.6,52.07 84.14,51.75 87,51.75 87.95,49.21 83.19,49.85 84.77,47.31 86.36,46.04 85.09,41.27 84.14,41.27 81.92,43.18 72.71,54.29 73.98,54.29 71.75,50.8 69.85,48.9 74.3,52.39 74.3,49.21 74.3,45.72 74.3,42.86 74.3,40.96 74.61,36.2 74.3,38.42 72.39,40.32 71.12,40.01 70.17,42.86 72.39,46.67 76.83,53.66 76.83,49.53 76.83,45.4 79.38,41.91 79.38,50.16 70.48,35.56 70.48,32.07 70.17,30.16 74.3,30.16 70.17,28.26 73.98,28.26 78.74,28.26 82.55,31.43 81.28,34.92 74.61,32.7 78.74,33.34 83.5,28.26 88.58,28.26 93.03,28.26 101.92,28.26 106.36,28.26 119.06,51.44 123.83,52.07 129.54,50.48 129.22,47.31 129.22,43.81 129.22,39.69 124.14,40.01 126.68,40.01 126.36,46.99 119.7,47.31 120.33,42.86 120.33,40.01 129.22,35.24 129.22,30.48 132.72,30.8 132.08,34.29 136.21,38.1 136.21,42.86 135.89,47.31 133.35,51.75 141.6,37.78 141.29,43.81 141.6,49.21 138.75,52.07 136.53,55.56 134.3,56.83 133.35,60.33 133.35,64.14 132.72,67.94 129.86,70.48 129.22,73.03 124.46,73.03 119.7,72.71 139.7,71.12 142.24,71.12 139.7,76.2 110.17,70.48 112.39,69.22 116.52,69.53 120.33,69.53 117.16,61.59 107.95,60.64 106.05,59.05 114.62,65.09 114.62,58.42 117.47,53.98 121.28,59.05 126.36,57.78 123.83,65.41 127.95,65.41 130.81,65.09 130.81,62.87 126.68,80.96 124.14,80.64 119.7,76.52 129.54,78.11 135.25,84.77 134.62,77.15 135.57,91.12 127.32,91.44 120.97,84.45 140.65,86.36 140.65,81.28 123.19,106.05 133.35,106.05 146.69,106.05 131.76,101.6 142.56,101.92 146.37,98.11 127.32,99.69 53.98,105.73 36.2,106.36 26.99,103.19 27.3,89.22 27.3,80.96 27.62,72.39 27.3,63.18 26.99,54.93 47.62,55.56 44.45,57.47 41.27,58.42 40.96,52.39 28.89,50.8 38.1,60.01 36.2,63.18 31.43,57.47 42.23,75.25 41.91,73.98 39.69,73.66 39.69,77.47 34.92,82.55 34.61,75.56 39.93,69.22 42.23,68.9 42.86,70.17 45.4,65.72 42.23,64.14 39.05,65.09 37.15,66.99 69.53,56.75 70.48,56.83 69.53,54.29 70.48,53.34 69.53,51.75 66.67,52.7 65.48,49.77 73.98,61.28 74.3,62.87 77.15,69.53 60.96,68.58 60.64,62.55 53.02,62.87 49.85,61.91 45.09,62.55 52.07,88.58 55.88,85.41 60.64,80.64 59.37,75.88 53.34,75.88 96.2,82.23 99.69,80.01 104.78,76.52 103.5,81.28 124.14,89.53 132.4,80.33 117.16,81.6 38.89,68.1
  pour Bottom (isolate 0.406, no thermals): 0,150 171,150 171,0 0,0
  pour Top (no thermals): 100.33,78.42 91.44,78.42 91.44,70.8 100.33,70.8
  pour Top (isolate 0.254, no thermals): 1.27,109.22 170.81,109.22 170.81,24.13 1.27,24.13
N$1
  Top 0.254: Q23.3 101.2,49.53 101.12,49.61 101.12,51.44 100.57,51.99 99.22,51.99 98.5,51.28 98.5,50.88 98.19,50.56 98.19,49.85 94.46,46.12 94.46,44.93 94.38,44.85 93.34,44.85 OK1.2
N$2
  Top 0.254: R2.1 35.96,41.91 35.96,45.09 Q1.3 34.69,45.09 33.81,45.96 33.81,46.51 33.89,46.59 33.89,48.58 34.53,49.21 Q2.1
N$3
  Top 0.254: OSC1.3 47.31,78.74 47.23,78.66 47.23,78.42 46.12,77.31 46.12,76.12 48.1,74.14 48.1,73.66 49.53,72.23 50.16,72.23 50.4,72.47 51.04,72.47 51.28,72.71 52.86,72.71 53.26,73.1 53.26,74.3 U1.59
N$4
  Top 0.254: R34.2 80.41,55.24 80.41,56.52 80.64,56.75 80.64,57.78 C2.1 81.28,57.78 81.36,57.86 81.36,60.25 | C1.1 81.28,60.33 81.36,60.25 | DC1.4 81.44,60.33 81.36,60.25
N$5
  Top 0.254: Q3.3 41.27,40.88 41.2,40.8 37.86,40.8 37.7,40.64 37.7,39.37 R4.1 37.7,39.29 37.7,38.1 37.78,38.02 38.58,38.02 38.89,37.7 41.04,37.7 41.12,37.78 42.31,37.78 Q4.1
N$6
  Top 0.254: C18.1 80.64,62.87 80.64,63.74 80.25,64.14 80.25,65.41 R5.1 80.25,65.48 80.25,66.04 83.82,66.04 DC1.2
N$7
  Top 0.254: 39.13,33.02 C4.2 | 39.13,33.02 38.73,33.42 37.47,33.42 R10.1 | ST3.2 39.05,30.8 39.05,32.94 39.13,33.02
N$8
  Top 0.254: R32.2 116.2,54.21 112.39,54.21 OK2.1
N$9
  Top 0.254: R7.1 44.85,41.91 44.85,45.09 Q5.3 43.58,45.09 42.7,45.96 42.7,46.51 42.78,46.59 42.78,48.58 43.42,49.21 Q6.1
N$10
  Top 0.254: R96.1 28.81,36.83 28.81,35.24 R94.2 28.57,35.16 29.92,35.16 30.32,35.56 C94.2 32.15,35.56 32.15,36.51 32.23,36.59 34.45,36.59 34.69,36.83 34.69,38.26 34.61,38.34 | Q32.3 32.31,38.73 32.46,38.58 32.54,38.58 32.62,38.66 34.29,38.66 34.61,38.34 | Q12.1 30.08,44.13 30.4,43.81 30.4,43.1 30.48,43.02 31.59,43.02 31.75,43.18 32.07,43.18 32.23,43.34 32.54,43.34 32.7,43.18 33.02,43.18 34.69,41.51 34.69,38.42 34.61,38.34
N$11
  Top 0.254: R1.1 37.7,36.83 37.7,35.24 R10.2 37.47,35.16 38.81,35.16 39.21,35.56 C3.2 41.04,35.56 41.04,36.51 41.12,36.59 43.34,36.59 43.58,36.83 43.58,38.26 43.5,38.34 | Q4.3 41.2,38.73 41.35,38.58 41.43,38.58 41.51,38.66 43.18,38.66 43.5,38.34 | Q1.1 37.94,44.13 38.97,44.13 39.29,43.81 39.29,43.1 39.37,43.02 40.48,43.02 40.64,43.18 40.96,43.18 41.12,43.34 41.43,43.34 41.59,43.18 41.91,43.18 43.58,41.51 43.58,38.42 43.5,38.34
N$12
  Top 0.254: Q7.3 50.16,40.88 50.09,40.8 46.91,40.8 46.59,40.48 46.59,39.37 R9.1 46.59,39.29 46.59,38.1 46.67,38.02 47.47,38.02 47.78,37.7 49.93,37.7 50.01,37.78 51.2,37.78 Q8.1
N$13
  Top 0.254: 48.02,33.02 C6.2 | 48.02,33.02 47.62,33.42 46.35,33.42 R15.1 | ST4.2 47.94,30.8 47.94,32.94 48.02,33.02
N$14
  Top 0.254: R6.1 46.59,36.83 46.59,35.24 R15.2 46.35,35.16 47.7,35.16 48.1,35.56 C5.2 49.93,35.56 49.93,36.51 50.01,36.59 52.23,36.59 52.47,36.83 52.47,38.26 52.39,38.34 | Q8.3 50.09,38.73 50.24,38.58 50.32,38.58 50.4,38.66 52.07,38.66 52.39,38.34 | Q5.1 46.83,44.13 47.86,44.13 48.18,43.81 48.18,43.1 48.26,43.02 49.37,43.02 49.53,43.18 49.85,43.18 50.01,43.34 50.32,43.34 50.48,43.18 50.8,43.18 52.47,41.51 52.47,38.42 52.39,38.34
N$15
  Top 0.254: 56.91,33.02 C8.2 | 56.91,33.02 56.52,33.42 55.24,33.42 R20.1 | ST5.2 56.83,30.8 56.83,32.94 56.91,33.02
N$16
  Top 0.254: R12.1 53.74,41.91 53.74,45.09 Q9.3 52.47,45.09 51.59,45.96 51.59,46.51 51.67,46.59 51.67,48.58 52.31,49.21 Q10.1
N$17
  Top 0.254: R27.1 100.09,42.55 100.09,45.72 Q22.3 98.74,45.72 98.66,45.8 98.66,50.32 98.82,50.48 99.85,50.48 Q23.1
N$18
  Top 0.254: OK2.4 107.31,44.85 106.05,44.85 105.89,44.69 104.78,44.69 R29.1 104.7,44.69 103.58,44.69 103.5,44.61 103.5,42.23 103.66,42.07 103.66,40.48 104.78,39.37 104.78,39.05 104.93,38.89 104.93,37.86 105.01,37.78 105.81,37.78 Q25.1
N$19
  Top 0.254: Q11.3 59.05,40.88 58.98,40.8 55.8,40.8 55.48,40.48 55.48,39.37 R14.1 55.48,39.29 55.48,38.1 55.56,38.02 56.36,38.02 56.67,37.7 58.82,37.7 58.9,37.78 60.09,37.78 Q13.1
N$20  (via drill 0.3)
  Top 0.61: IC1.1 98.19,82.31 98.19,82.87 C20.1 101.84,82.87 103.66,82.87 103.98,83.19 C22.+ 130.18,83.19 135.1,88.11 136.05,88.11 v136.21,88.27 | v137.64,88.27 137.56,88.34 137.56,88.82 138.43,89.69 139.7,89.69 L1.1
  Bottom 0.61: v136.21,88.27 v137.64,88.27
N$21
  Top 0.254: R11.1 55.48,36.83 55.48,35.24 R20.2 55.24,35.16 56.59,35.16 56.99,35.56 C7.2 58.82,35.56 58.82,36.51 58.9,36.59 61.12,36.59 61.36,36.83 61.36,38.26 61.28,38.34 | Q13.3 58.98,38.73 59.13,38.58 59.21,38.58 59.29,38.66 60.96,38.66 61.28,38.34 | Q9.1 56.75,44.13 57.07,43.81 57.07,43.1 57.15,43.02 58.26,43.02 58.42,43.18 58.74,43.18 58.9,43.34 59.21,43.34 59.37,43.18 59.69,43.18 61.36,41.51 61.36,38.42 61.28,38.34
N$22
  Top 0.254: 65.8,33.02 C10.2 67.71,33.02 67.71,32.07 67.79,31.99 68.9,31.99 69.85,31.04 72.39,31.04 D1.C | 65.8,33.02 65.41,33.42 64.14,33.42 R25.1 | ST6.2 65.41,32.62 65.8,33.02
N$23
  Top 0.254: R17.1 62.63,41.91 62.63,45.09 Q14.3 61.36,45.09 60.48,45.96 60.48,46.51 60.56,46.59 60.56,48.58 61.2,49.21 Q15.1
N$24
  Top 0.254: R16.1 64.37,36.83 64.37,35.24 R25.2 64.14,35.16 65.48,35.16 65.88,35.56 C9.2 67.71,35.56 67.71,36.51 67.94,36.75 70.17,36.75 70.33,36.91 70.33,38.02 70.41,38.1 | Q17.3 67.87,38.73 68.02,38.58 68.1,38.58 68.18,38.66 69.85,38.66 70.17,38.34 | 70.41,38.1 70.17,38.34 | 70.41,38.1 71.04,38.1 71.12,38.02 72.39,38.02 D3.C | Q14.1 64.61,44.13 65.64,44.13 65.96,43.81 65.96,43.1 66.04,43.02 67.15,43.02 67.31,43.18 67.63,43.18 67.79,43.34 68.1,43.34 68.26,43.18 68.58,43.18 70.25,41.51 70.25,38.42 70.17,38.34
N$25
  Top 0.254: 84.22,33.02 C15.2 86.12,33.02 86.12,32.07 86.2,31.99 87.31,31.99 88.27,31.04 90.81,31.04 D5.C | 84.22,33.02 83.82,33.42 82.55,33.42 R30.1 | ST7.2 83.82,32.62 84.22,33.02
N$26
  Top 0.254: Q16.3 67.94,40.88 67.87,40.8 64.69,40.8 64.37,40.48 64.37,39.37 R19.1 64.37,39.29 64.37,38.1 64.45,38.02 65.25,38.02 65.56,37.7 67.71,37.7 67.79,37.78 68.98,37.78 Q17.1
N$27  (via drill 0.3)
  Top 0.254: v63.1,104.62 62.39,105.33 61.75,105.33 61.36,104.93 61.36,104.62 60.88,104.14 60.88,103.5 59.61,102.23 54.13,102.23 53.9,102.47 34.77,102.47 27.86,95.57 27.86,94.93 27.78,94.85 26.67,94.85 R41.1 | v64.14,103.58 66.83,103.58 67.63,104.38 73.34,104.38 75.09,102.63 v75.41,102.63 | v73.98,101.2 73.98,100.25 v75.01,99.22 | v77.39,98.35 77.39,99.62 JP6.1
  Bottom 0.254: v64.14,103.58 v63.1,104.62 | v73.98,101.2 v75.41,102.63 | v75.01,99.22 76.52,99.22 v77.39,98.35
N$28
  Top 0.254: R21.1 82.79,36.83 82.79,35.24 R30.2 82.55,35.16 83.9,35.16 84.3,35.56 C14.2 86.12,35.56 86.12,36.51 86.36,36.75 88.58,36.75 88.74,36.91 88.74,38.02 88.82,38.1 | Q21.3 86.28,38.73 86.44,38.58 86.52,38.58 86.6,38.66 88.27,38.66 88.58,38.34 | 88.82,38.1 88.58,38.34 | 88.82,38.1 89.46,38.1 89.53,38.02 90.81,38.02 D7.C | Q18.1 84.06,44.13 84.38,43.81 84.38,43.1 84.45,43.02 85.57,43.02 85.72,43.18 86.04,43.18 86.2,43.34 86.52,43.34 86.68,43.18 87,43.18 88.66,41.51 88.66,38.42 88.58,38.34
N$29
  Top 0.254: 102.63,33.02 C17.2 104.54,33.02 104.54,32.07 104.62,31.99 105.97,31.99 107.55,30.4 109.22,30.4 D15.C | 102.63,33.02 102.23,33.42 100.97,33.42 R33.1 | ST8.2 102.23,32.62 102.63,33.02
N$30
  Top 0.254: R22.1 81.04,41.91 81.04,45.09 Q18.3 79.61,45.09 78.98,45.72 78.98,48.42 79.77,49.21 80.8,49.21 Q19.1
N$31
  Top 0.254: 101.84,38.5 101.84,38.58 101.92,38.66 102.39,38.66 102.47,38.73 Q25.3 | 101.84,38.5 101.84,37.47 R26.1 101.84,37.39 101.84,35.16 | Q22.1 102,44.77 101.2,44.77 101.12,44.69 101.12,43.42 100.97,43.26 100.97,41.83 101.28,41.51 101.28,41.04 100.97,40.72 100.97,39.29 101.76,38.5 101.84,38.5 | 101.84,35.16 102.31,35.16 102.71,35.56 C16.2 104.54,35.56 104.54,36.51 104.62,36.59 106.84,36.59 107.63,37.39 109.22,37.39 D17.C | 101.84,35.16 100.97,35.16 R33.2
N$32  (via drill 0.3)
  Top 0.254: v62.07,104.62 61.36,103.9 61.36,103.27 59.85,101.76 53.9,101.76 53.66,102 35,102 30.4,97.39 30.4,94.93 30.32,94.85 29.21,94.85 R42.1 | v63.1,105.65 64.77,105.65 64.93,105.81 75.09,105.81 v75.33,106.05 | v77.47,103.9 78.26,103.9 78.74,103.43 78.74,101.92 78.98,101.68 78.98,101.36 80.01,100.33 JP6.3
  Bottom 0.254: v63.1,105.65 v62.07,104.62 | v77.47,103.9 v75.33,106.05
N$33
  Top 0.254: Q20.3 86.36,40.88 85.65,40.16 82.79,40.16 82.79,39.37 R24.1 82.79,39.29 82.79,38.1 82.87,38.02 83.66,38.02 83.98,37.7 86.12,37.7 86.2,37.78 87.39,37.78 Q21.1
N$34
  Top 0.406: JP1.1 140.97,73.58 140.81,73.74 139.7,73.74 D31.2
N$35
  Top 0.254: D15.A D16.A
N$36
  Top 0.254: D17.A 109.22,41.35 113.67,41.35 D18.A
N$37
  Top 0.254: C24.2 119.38,33.02 119.46,33.1 119.46,33.42 120.02,33.42 R35.1 120.09,33.42 120.65,33.42 | JP3.3 120.65,33.42 | 120.65,33.42 121.05,33.42 121.13,33.5 121.13,36.12 119.22,38.02 118.11,38.02 D19.C
N$38
  Top 0.254: R35.2 120.02,35.16 119.46,35.16 119.46,35.48 119.38,35.56 C23.2 117.71,35.56 117.71,36.04 117.08,36.67 116.92,36.67 116.6,36.99 116.6,44.77 116.84,45.01 118.11,45.01 D21.C 118.19,45.01 119.62,45.01 122.08,47.47 123.98,47.47 124.54,48.02 124.54,53.42 124.46,53.5 IC12.13 124.46,55.96 124.14,56.28 122.87,56.28 119.38,59.77 IC12.8
N$39
  Top 0.254: D19.A 118.11,41.99 122.56,41.99 D20.A
N$40
  Top 0.254: D21.A 118.11,48.97 122.56,48.97 D22.A
N$41
  Top 0.254: 123.19,33.42 123.67,33.42 123.9,33.66 C26.2 124.86,33.66 124.86,32.7 124.94,32.62 127,32.62 127.71,33.34 127.71,38.02 127,38.02 D23.C | 123.19,33.42 122.56,33.42 R36.1 | JP3.2 123.19,33.42
N$42
  Top 0.254: 138.43,33.66 C28.2 | 138.43,33.66 138.51,33.73 138.51,34.05 139.06,34.05 R37.1 | JP4.3 138.43,33.66
N$43
  Top 0.254: D23.A 127,41.99 131.44,41.99 D24.A
N$44
  Top 0.254: D25.A 127,48.97 131.44,48.97 D26.A
N$45
  Top 0.254: IC12.3 125.73,61.99 126.13,62.39 C64.1
N$46
  Top 0.254: IC12.1 128.27,61.99 127.87,62.39 C64.2
N$47
  Top 0.254: IC12.4 124.46,62.07 124.7,62.31 C65.2
N$48
  Top 0.254: IC12.5 123.19,62.07 122.95,62.31 C65.1
N$49
  Top 0.254: IC12.2 127,59.61 127.79,58.82 C58.1
N$50
  Top 0.254: IC12.6 121.92,61.99 121.52,62.39 C57.2
N$51
  Top 0.254: OK4.4 122.56,67.07 121.28,67.07 118.51,64.29 118.51,59.37 118.59,59.29 119.14,59.29 121.92,56.52 IC12.11 121.92,53.74 121.84,53.66 120.73,53.66 120.65,53.74 IC12.10
N$52  (via drill 0.3)
  Top 0.254: v114.14,56.36 113.9,56.12 111.2,56.12 110.97,56.36 110.97,57.47 110.89,57.55 109.86,57.55 OK3.2 | v115.17,55.32 117.16,55.32 118.51,53.98 118.51,53.26 118.59,53.18 122.87,53.18 123.19,53.5 IC12.12
  Bottom 0.254: v115.17,55.32 v114.14,56.36
N$53  (via drill 0.3)
  Top 0.254: C27.2 138.43,36.2 138.51,36.12 138.51,35.8 139.06,35.8 R37.2 139.14,35.8 139.7,35.8 139.7,48.1 131.84,55.96 131.84,65.56 126.21,71.2 122.63,71.2 122.56,71.28 121.52,71.28 120.97,70.72 111.68,70.72 110.49,71.91 IC2.13 110.49,74.37 v109.93,74.93 | IC2.8 105.41,78.18 107.63,75.96 v108.9,75.96
  Bottom 0.254: v109.93,74.93 v108.9,75.96
N$54
  Top 0.254: 125.33,35.56 125.33,35.08 124.94,34.69 123.59,34.69 123.19,35.08 123.19,35.16 122.56,35.16 R36.2 | C25.2 125.33,35.56 | 125.89,45.01 127,45.01 D25.C | 125.89,45.01 125.02,45.88 125.02,52.78 125.73,53.5 IC12.14 | 125.33,35.56 125.33,44.45 125.89,45.01
N$55  (via drill 0.3)
  Top 0.254: v50.8,99.85 50.56,100.09 48.9,100.09 44.61,95.81 44.61,95.17 44.29,94.85 43.18,94.85 R43.1 | v51.91,100.81 52.15,101.04 53.18,101.04 53.9,100.33 64.29,100.33 67.87,103.9 73.1,103.9 76.04,100.97 78.66,100.97 78.74,100.89 78.74,98.42 v80.33,96.84 | v81.36,95.81 81.36,96.12 81.76,96.52 81.76,98.9 JP6.5
  Bottom 0.254: v50.8,99.85 51.75,100.81 v51.91,100.81 | v81.36,95.81 v80.33,96.84
N$56  (via drill 0.3)
  Top 0.254: v79.61,96.12 78.58,96.12 76.2,98.5 76.2,100.09 72.87,103.43 68.1,103.43 64.53,99.85 52.94,99.85 47.94,94.85 45.72,94.85 R44.1 | v80.64,95.09 81.68,95.09 82.07,95.49 82.07,96.12 82.23,96.28 82.23,96.84 JP6.7
  Bottom 0.254: v80.64,95.09 v79.61,96.12
N$57
  Top 0.254: C30.2 141.6,33.66 141.53,33.73 141.53,34.05 140.97,34.05 R38.1 140.89,34.05 140.49,34.05 140.49,30.96 JP4.2
N$58
  Top 0.254: JP6.9 87.63,94.3 87,93.66 85.65,93.66 85.57,93.58 80.49,93.58 80.09,93.98 71.2,93.98 70.8,93.58 69.06,93.58 67.79,94.85 60.96,94.85 R45.1
N$59  (via drill 0.3)
  Top 0.254: v75.49,91.2 75.49,91.44 74.53,92.39 71.2,92.39 70.64,93.11 68.82,93.11 67.55,94.38 62.07,94.38 61.67,93.98 60.25,93.98 59.85,94.38 59.85,94.54 59.53,94.85 58.42,94.85 R46.1 | v78.03,90.33 78.34,90.65 81.12,90.65 81.68,91.2 83.42,91.2 v83.82,90.81 | v85.96,92.95 86.2,93.19 87.23,93.19 88.11,94.06 88.11,97.63 JP6.11
  Bottom 0.254: v75.49,91.2 77.15,91.2 v78.03,90.33 | v85.96,92.95 v83.82,90.81
N$60
  Top 0.254: IC2.3 111.76,80.49 112.08,80.8 112.71,80.8 112.79,80.88 C31.1
N$61
  Top 0.254: IC2.1 114.3,80.49 114.54,80.72 C31.2
N$62
  Top 0.254: IC2.4 110.49,80.49 110.73,80.72 C32.2
N$63
  Top 0.254: IC2.5 109.22,80.49 108.98,80.72 C32.1
N$64
  Top 0.254: IC2.2 113.03,78.03 113.35,77.71 115.09,77.71 115.25,77.87 C33.1
N$65
  Top 0.254: IC2.6 107.95,80.49 107.63,80.8 107,80.8 106.92,80.88 C34.2
N$66  (via drill 0.3)
  Top 0.254: IC2.10 106.68,74.22 106.76,74.3 107.87,74.3 107.95,74.22 IC2.11 107.95,71.44 111.28,68.1 111.28,66.99 111.36,66.91 111.92,66.91 OK3.4 112.39,66.91 112,66.91 v112,64.61 | v60.96,54.05 61.2,54.29 61.2,54.93 59.61,56.52 59.61,59.05 U1.30 | v62.39,52.63 62.39,52.94 63.26,53.82 65.56,53.82 69.77,58.02 v71.2,58.02 | v72.87,56.91 73.1,56.67 76.2,56.67 79.45,53.42 v79.45,53.1 | v80.49,54.13 80.88,54.13 81.28,54.53 81.28,55.96 82.23,56.91 87.39,56.91 90.57,60.09 90.57,61.91 90.96,62.31 92.95,62.31 96.44,58.82 100.89,58.82 101.12,58.58 101.76,58.58 105.41,62.23 108.19,62.23 108.51,62.55 109.62,62.55 110.65,63.58 v110.97,63.58
  Bottom 0.254: v62.39,52.63 v60.96,54.05 | v71.2,58.02 71.75,58.02 v72.87,56.91 | v80.49,54.13 v79.45,53.1 | v112,64.61 v110.97,63.58
N$67  (via drill 0.3)
  Top 0.254: v117,104.78 117,105.09 114.86,107.24 77.55,107.24 75.64,105.33 65.17,105.33 65.01,105.17 64.69,105.17 63.42,103.9 62.71,103.9 60.09,101.28 53.66,101.28 53.42,101.52 38.34,101.52 35.72,98.9 35.72,90.49 35.8,90.41 35.8,88.19 33.02,85.41 33.02,74.45 34.77,72.71 34.77,69.85 34.45,69.53 34.45,67.87 42.62,59.69 48.1,59.69 48.74,60.33 60.33,60.33 60.48,60.17 60.48,59.05 U1.31 | v118.03,105.81 119.06,105.81 119.46,105.41 119.46,104.78 126.6,97.63 132.08,97.63 133.11,96.6 137.48,96.6 138.27,97.39 140.1,97.39 140.81,98.11 143.11,98.11 143.75,97.47 143.75,88.9 142.4,87.55 139.62,87.55 138.67,86.6 v138.67,86.28 | v137.64,87.31 137,87.31 136.68,87 135.65,87 126.36,77.71 126.29,77.71 125.49,77.63 | 125.49,77.63 125.49,76.44 125.09,76.44 OK4.2 | IC2.12 109.22,75.25 110.17,76.2 113.74,76.2 114.38,75.56 116.6,75.56 118.75,77.71 126.13,77.71 125.49,77.63
  Bottom 0.254: v118.03,105.81 v117,104.78 | v137.64,87.31 v138.67,86.28
N$68
  Top 0.254: C29.2 142.16,36.2 142.16,35.88 142.08,35.8 140.97,35.8 R38.2 140.89,35.8 140.18,35.8 140.18,48.34 132.32,56.2 132.32,65.8 126.44,71.68 122.87,71.68 122.79,71.75 121.28,71.75 120.73,71.2 115.81,71.2 115.17,71.83 115.17,74.61 115.09,74.69 112.08,74.69 111.76,74.37 IC2.14
N$69  (via drill 0.3)
  Top 0.254: v78.26,94.69 78.11,94.85 76.83,94.85 R47.1 | v78.26,93.27 78.26,92.15 78.34,92.08 80.41,92.08 80.96,92.63 84.45,92.63 87.07,90.01 v87.15,90.01 | v88.19,91.04 88.74,91.6 88.74,92 v90.41,93.66 | v91.44,94.69 91.2,94.93 91.2,96.12 91.12,96.2 91.12,97.47 91.92,98.27 91.92,98.9 JP6.13
  Bottom 0.254: v78.26,93.27 v78.26,94.69 | v88.19,91.04 v87.15,90.01 | v91.44,94.69 v90.41,93.66
N$70
  Top 0.254: R39.1 104.78,56.75 105.89,56.75 105.97,56.83 105.97,57.47 106.05,57.55 107.31,57.55 OK3.1
N$71
  Top 0.254: R40.1 131.44,76.44 127.64,76.44 OK4.1
N$72  (via drill 0.3)
  Top 0.254: v97.55,102.55 97.23,102.55 95.01,104.78 91.84,104.78 91.44,104.38 91.44,101.6 91.04,101.2 90.73,101.2 90.49,100.97 81.36,100.97 81.28,100.89 81.28,96.76 79.38,94.85 R48.1 | v96.52,101.52 96.52,100.97 JP6.15
  Bottom 0.254: v96.52,101.52 v97.55,102.55
N$73
  Top 0.254: JP6.16 93.98,100.97 93.98,95.01 94.14,94.85 95.25,94.85 R49.1
N$74
  Top 0.254: JP6.14 92.71,102.16 91.44,100.89 91.44,98.5 90.65,97.71 90.65,95.96 90.73,95.89 90.73,94.38 91.52,93.58 94.14,93.58 94.54,93.98 95.96,93.98 96.36,94.38 96.36,94.54 96.68,94.85 97.79,94.85 R50.1
N$75  (via drill 0.3)
  Top 0.254: v101.84,99.85 106.84,94.85 111.76,94.85 R51.1 | v100.81,100.89 100.17,100.89 v99.77,101.28 | v98.74,102.31 98.27,102.79 98.27,102.87 97.87,103.27 97.23,103.27 95.25,105.25 91.6,105.25 90.96,104.62 90.96,103.03 JP6.12
  Bottom 0.254: v100.81,100.89 v101.84,99.85 | v98.74,102.31 v99.77,101.28
N$76  (via drill 0.3)
  Top 0.254: v115.25,103.03 115.25,94.93 115.17,94.85 114.3,94.85 R52.1 | v116.28,104.06 116.28,105.09 114.62,106.76 97.55,106.76 v96.52,105.73 | v94.38,103.58 94.14,103.82 93.27,103.82 v93.03,103.58 | v90.25,103.58 88.98,103.58 JP6.10
  Bottom 0.254: v116.28,104.06 v115.25,103.03 | v94.38,103.58 v96.52,105.73 | v93.03,103.58 92.71,103.58 92.47,103.35 92.23,103.35 92.15,103.27 91.6,103.27 91.28,103.58 v90.25,103.58
N$77  (via drill 0.3)
  Top 0.254: v76.2,106.92 76.52,106.92 77.31,107.71 115.09,107.71 126.68,96.12 128.27,96.12 R53.1 | v77.71,105.65 77.95,105.41 81.92,105.41 JP6.8
  Bottom 0.254: v76.2,106.92 76.44,106.92 v77.71,105.65
N$78  (via drill 0.3)
  Top 0.254: v77.55,92 77.95,91.6 80.64,91.6 81.2,92.15 84.22,92.15 86.44,89.93 86.44,89.69 86.84,89.3 88.19,89.3 89.06,88.42 90.01,88.42 91.36,87.07 94.93,87.07 95.17,86.84 95.49,86.84 96.04,86.28 96.6,86.28 97.39,85.49 102.08,85.49 103.27,84.3 117.4,84.3 118.27,85.17 118.27,85.8 125.81,93.34 129.3,93.34 129.46,93.5 129.46,95.89 129.7,96.12 130.81,96.12 R54.1 | v75.72,94.69 75.72,99.85 75.01,100.57 v74.69,100.57 | v76.12,102 76.12,103.58 77.47,104.93 81.68,104.93 82.55,104.06 JP6.6
  Bottom 0.254: v77.55,92 77.55,92.87 v75.72,94.69 | v76.12,102 v74.69,100.57
N$79  (via drill 0.3)
  Top 0.254: v118.75,105.09 118.75,104.78 126.36,97.16 131.84,97.16 132.87,96.12 139.06,96.12 R55.1 | v117.71,104.06 117.32,104.06 116.6,103.35 115.97,103.35 114.86,104.46 114.86,105.09 114.14,105.81 104.38,105.81 v102.08,103.5 | v101.04,102.47 99.93,102.47 99.06,101.6 97.47,101.6 94.77,104.3 92.39,104.3 v92.15,104.06 | v90.73,105.49 90.41,105.81 83.74,105.81 v83.19,105.25 | v81.76,103.82 81.6,103.82 JP6.4
  Bottom 0.254: v117.71,104.06 v118.75,105.09 | v101.04,102.47 v102.08,103.5 | v90.73,105.49 v92.15,104.06 | v81.76,103.82 v83.19,105.25
N$80  (via drill 0.3)
  Top 0.254: v142.56,89.53 142.8,89.77 142.8,96.04 142.72,96.12 141.6,96.12 R56.1 | v143.99,88.11 143.99,88.42 144.22,88.66 144.22,97.71 143.35,98.58 140.57,98.58 139.86,97.87 138.03,97.87 137.24,97.08 133.35,97.08 132.32,98.11 126.84,98.11 119.94,105.01 119.94,105.65 119.3,106.28 118.59,106.28 118.35,106.52 v117.32,106.52 | v115.57,104.78 115.57,105.09 114.38,106.28 97.79,106.28 97.55,106.05 v97.55,105.73 | v94.22,105.97 93.9,106.28 82.87,106.28 v82.47,105.89 | v80.8,104.22 80.57,104.46 79.69,104.46 v79.22,103.98
  Bottom 0.254: v143.99,88.11 v142.56,89.53 | v115.57,104.78 v117.32,106.52 | v97.55,105.73 96.84,106.44 94.69,106.44 v94.22,105.97 | v80.8,104.22 v82.47,105.89 | JP6.2 v79.22,103.98
N$81  (via drill 0.3)
  Top 0.254: v32.62,86.04 32.54,86.12 32.54,90.17 30.64,92.08 28.18,92.08 27.86,92.39 27.86,93.03 27.78,93.11 26.67,93.11 R41.2 | v34.21,84.45 34.85,84.45 45.01,74.3 45.88,74.3 46.35,73.82 v47.39,73.82 | v49.85,72.95 50.8,72.95 50.88,73.03 50.88,74.3 U1.62
  Bottom 0.254: v34.21,84.45 v32.62,86.04 | v47.39,73.82 48.97,73.82 v49.85,72.95
N$82  (via drill 0.3)
  Top 0.254: v33.26,86.76 33.02,87 33.02,90.41 30.32,93.11 29.21,93.11 R42.2 | v34.69,85.33 45.24,74.77 v46.43,74.77 | v47.47,75.8 47.7,75.8 v48.9,76.99 | v49.93,75.96 49.93,75.64 50.01,75.56 50.01,74.3 U1.63
  Bottom 0.254: v34.69,85.33 v33.26,86.76 | v47.47,75.8 v46.43,74.77 | v49.93,75.96 v48.9,76.99
N$83
  Top 0.254: R43.2 43.18,93.11 43.89,93.11 44.53,93.74 44.77,93.74 45.01,93.98 46.43,93.98 50.96,89.46 50.96,79.45 50.09,78.58 50.09,77.15 49.21,76.28 49.21,74.3 U1.64
N$84  (via drill 0.3)
  Top 0.254: v40.16,80.96 40.16,82.71 44.29,86.84 44.29,92.79 44.61,93.11 45.72,93.11 R44.2 | v38.73,79.53 39.05,79.53 43.42,75.17 v43.42,73.5 | v44.61,72.63 44.85,72.39 46.04,72.39 46.35,72.71 47.62,72.71 U1.1
  Bottom 0.254: v38.73,79.53 v40.16,80.96 | v43.42,73.5 43.74,73.5 v44.61,72.63
N$85  (via drill 0.3)
  Top 0.254: v52.86,98.74 52.94,98.74 57.71,93.98 59.13,93.98 59.37,93.74 59.61,93.74 60.25,93.11 60.96,93.11 R45.2 | v51.83,99.77 51.51,100.09 51.51,100.17 50.64,101.04 38.58,101.04 36.2,98.66 36.2,90.73 36.27,90.65 36.27,87.95 33.5,85.17 33.5,74.69 35.24,72.95 35.24,72.15 36.75,70.64 38.89,70.64 40.16,71.91 47.62,71.91 U1.2
  Bottom 0.254: v51.83,99.77 v52.86,98.74
N$86  (via drill 0.3)
  Top 0.254: v60.17,84.3 59.85,84.61 59.85,92.79 59.53,93.11 58.42,93.11 R46.2 | v59.13,83.26 59.13,79.53 58.74,79.14 57.23,79.14 56.12,78.03 56.12,75.88 v56.36,75.64 | v53.98,72.95 53.82,72.95 53.1,72.23 51.51,72.23 51.28,71.99 50.64,71.99 50.4,71.75 49.61,71.75 48.9,71.04 47.62,71.04 U1.3
  Bottom 0.254: v59.13,83.26 v60.17,84.3 | v56.36,75.64 56.36,75.33 v53.98,72.95
N$87  (via drill 0.3)
  Top 0.254: v75.72,93.11 76.83,93.11 R47.2 | v74.22,91.6 74.22,86.2 68.42,80.41 64.77,80.41 v64.69,80.49 | v63.26,79.06 61.44,79.06 60.88,78.5 60.88,77.87 61.28,77.47 61.28,75.8 v61.12,75.64 | v59.29,72.95 59.29,72.15 56.83,69.69 50.56,69.69 50.09,70.17 49.05,70.17 48.97,70.25 47.62,70.25 U1.4
  Bottom 0.254: v74.22,91.6 v75.72,93.11 | v63.26,79.06 v64.69,80.49 | v61.12,75.64 61.12,74.77 v59.29,72.95
N$88  (via drill 0.3)
  Top 0.254: v65.48,104.62 65.72,104.85 75.88,104.85 77.79,106.76 94.46,106.76 97.47,103.74 98.11,103.74 98.66,103.19 101.36,103.19 101.76,102.79 101.76,100.81 101.12,100.17 101.12,94.38 98.82,92.08 97.31,92.08 94.77,89.53 94.46,89.53 93.5,88.58 90.57,88.58 90.25,88.9 89.3,88.9 87.47,90.73 87.07,90.73 84.69,93.11 79.38,93.11 R48.2 | v63.74,106.36 62.07,106.36 60.88,105.17 60.88,104.85 60.4,104.38 60.4,103.74 59.37,102.71 54.37,102.71 54.13,102.95 34.53,102.95 27.46,95.89 25.64,95.89 25.56,95.81 25.56,92.15 25.64,92.08 27.46,92.08 27.94,91.6 30.4,91.6 32.07,89.93 32.07,86.52 31.91,86.36 31.91,74.85 34.29,72.47 34.29,70.09 33.97,69.77 33.97,67.31 v34.13,67.15 | v35.16,68.18 37.39,68.18 v38.1,68.9 | v39.13,69.93 39.13,70.17 40.4,71.44 44.37,71.44 46.35,69.45 47.62,69.45 U1.5
  Bottom 0.254: v63.74,106.36 v65.48,104.62 | v35.16,68.18 v34.13,67.15 | v39.13,69.93 v38.1,68.9
N$89  (via drill 0.3)
  Top 0.254: v88.98,90.25 88.98,91.12 89.22,91.36 89.22,91.76 90.41,92.95 90.73,92.95 90.88,93.11 95.25,93.11 R49.2 | v87.31,88.58 87.07,88.82 86.6,88.82 85.96,89.46 85.96,89.69 83.98,91.68 81.44,91.68 80.88,91.12 77.79,91.12 77.31,90.65 77.31,89.06 v77.55,88.82 | v75.49,86.76 68.66,79.93 67.07,79.93 62.39,75.25 v62.07,75.25 | v60.33,72.95 60.33,72.47 57.07,69.22 49.53,69.22 48.97,68.66 47.62,68.66 U1.6
  Bottom 0.254: v87.31,88.58 v88.98,90.25 | v75.49,86.76 v77.55,88.82 | v62.07,75.25 62.07,74.69 v60.33,72.95
N$90  (via drill 0.3)
  Top 0.254: v89.69,89.61 89.93,89.38 90.49,89.38 90.81,89.06 93.27,89.06 94.22,90.01 94.54,90.01 96.6,92.08 96.6,93.03 96.68,93.11 97.79,93.11 R50.2 | v88.27,88.19 88.27,79.22 v85.41,76.36 | v84.38,75.33 82.39,73.34 78.03,73.34 77.71,73.66 77.71,73.98 v76.99,74.69 | v75.41,74.69 75.09,74.69 74.77,75.01 64.29,75.01 63.1,73.82 v63.1,73.5 | v61.52,71.91 61.2,71.91 55.8,66.52 53.5,66.52 52.55,67.63 51.99,68.26 49.29,68.26 48.9,67.87 U1.7
  Bottom 0.254: v88.27,88.19 v89.69,89.61 | v84.38,75.33 v85.41,76.36 | v75.41,74.69 v76.99,74.69 | v61.52,71.91 v63.1,73.5
N$91  (via drill 0.3)
  Top 0.254: v96.6,87.47 96.84,87.47 97.87,86.44 100.41,86.44 107.08,93.11 111.76,93.11 R51.2 | v95.17,86.12 94.69,86.6 91.36,86.6 88.74,83.98 88.74,78.98 87.15,77.39 87.15,75.41 v86.76,75.01 | v85.33,73.58 84.61,72.87 77.79,72.87 v76.99,73.66 | v75.41,73.66 74.53,74.53 64.53,74.53 64.06,74.06 v64.06,73.74 | v62.15,73.74 60.88,72.47 60.88,72.31 56.83,68.26 v53.66,68.26 | v52.23,66.91 51.99,67.07 U1.8
  Bottom 0.254: v96.6,87.47 95.25,86.12 v95.17,86.12 | v85.33,73.58 v86.76,75.01 | v75.41,73.66 v76.99,73.66 | v64.06,73.74 63.9,73.74 63.42,74.22 62.63,74.22 v62.15,73.74 | v53.66,68.26 52.31,66.91 v52.23,66.91
N$92  (via drill 0.3)
  Top 0.254: v94.54,87.79 95.01,88.27 96.84,88.27 97.31,87.79 97.31,87.71 98.11,86.92 100.17,86.92 106.84,93.58 110.65,93.58 111.05,93.98 112.47,93.98 112.87,93.58 112.87,93.42 113.19,93.11 114.3,93.11 R52.2 | v93.11,85.88 92.87,86.12 91.6,86.12 89.3,83.82 89.3,78.82 87.63,77.15 87.63,74.37 v87.55,74.3 | v86.12,72.87 85.65,72.39 77.23,72.39 v76.99,72.63 | v75.41,72.63 74.69,73.34 74.69,73.66 74.3,74.06 65.41,74.06 v65.01,73.66 | v61.52,70.96 60.96,70.96 56.83,66.83 56.83,66.2 55.17,64.53 50.72,64.53 48.97,66.28 U1.9
  Bottom 0.254: v94.54,87.79 94.54,87.31 v93.11,85.88 | v86.12,72.87 v87.55,74.3 | v75.41,72.63 v76.99,72.63 | v65.01,73.66 62.31,70.96 v61.52,70.96
N$93  (via drill 0.3)
  Top 0.254: v95.49,87.55 96.28,86.76 96.84,86.76 97.63,85.96 102.31,85.96 103.5,84.77 117.16,84.77 117.79,85.41 117.79,86.04 126.13,94.38 128.27,94.38 R53.2 | v94.22,85.88 94.22,84.93 95.01,84.14 v95.01,80.88 | v93.9,79.77 93.66,79.53 90.73,79.53 88.11,76.91 88.11,76.2 88.34,75.96 88.34,73.74 v88.19,73.58 | v86.76,72.15 86.12,72.15 85.88,71.91 77.23,71.91 v76.99,71.68 | v75.41,71.68 68.34,71.68 67.31,72.71 v67.31,73.03 | v66.28,71.99 66.04,72.23 64.61,72.23 v64.21,71.83 | v61.52,69.93 60.64,69.93 57.31,66.6 57.31,65.96 55.48,64.06 50.48,64.06 48.97,65.56 48.9,65.48 U1.10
